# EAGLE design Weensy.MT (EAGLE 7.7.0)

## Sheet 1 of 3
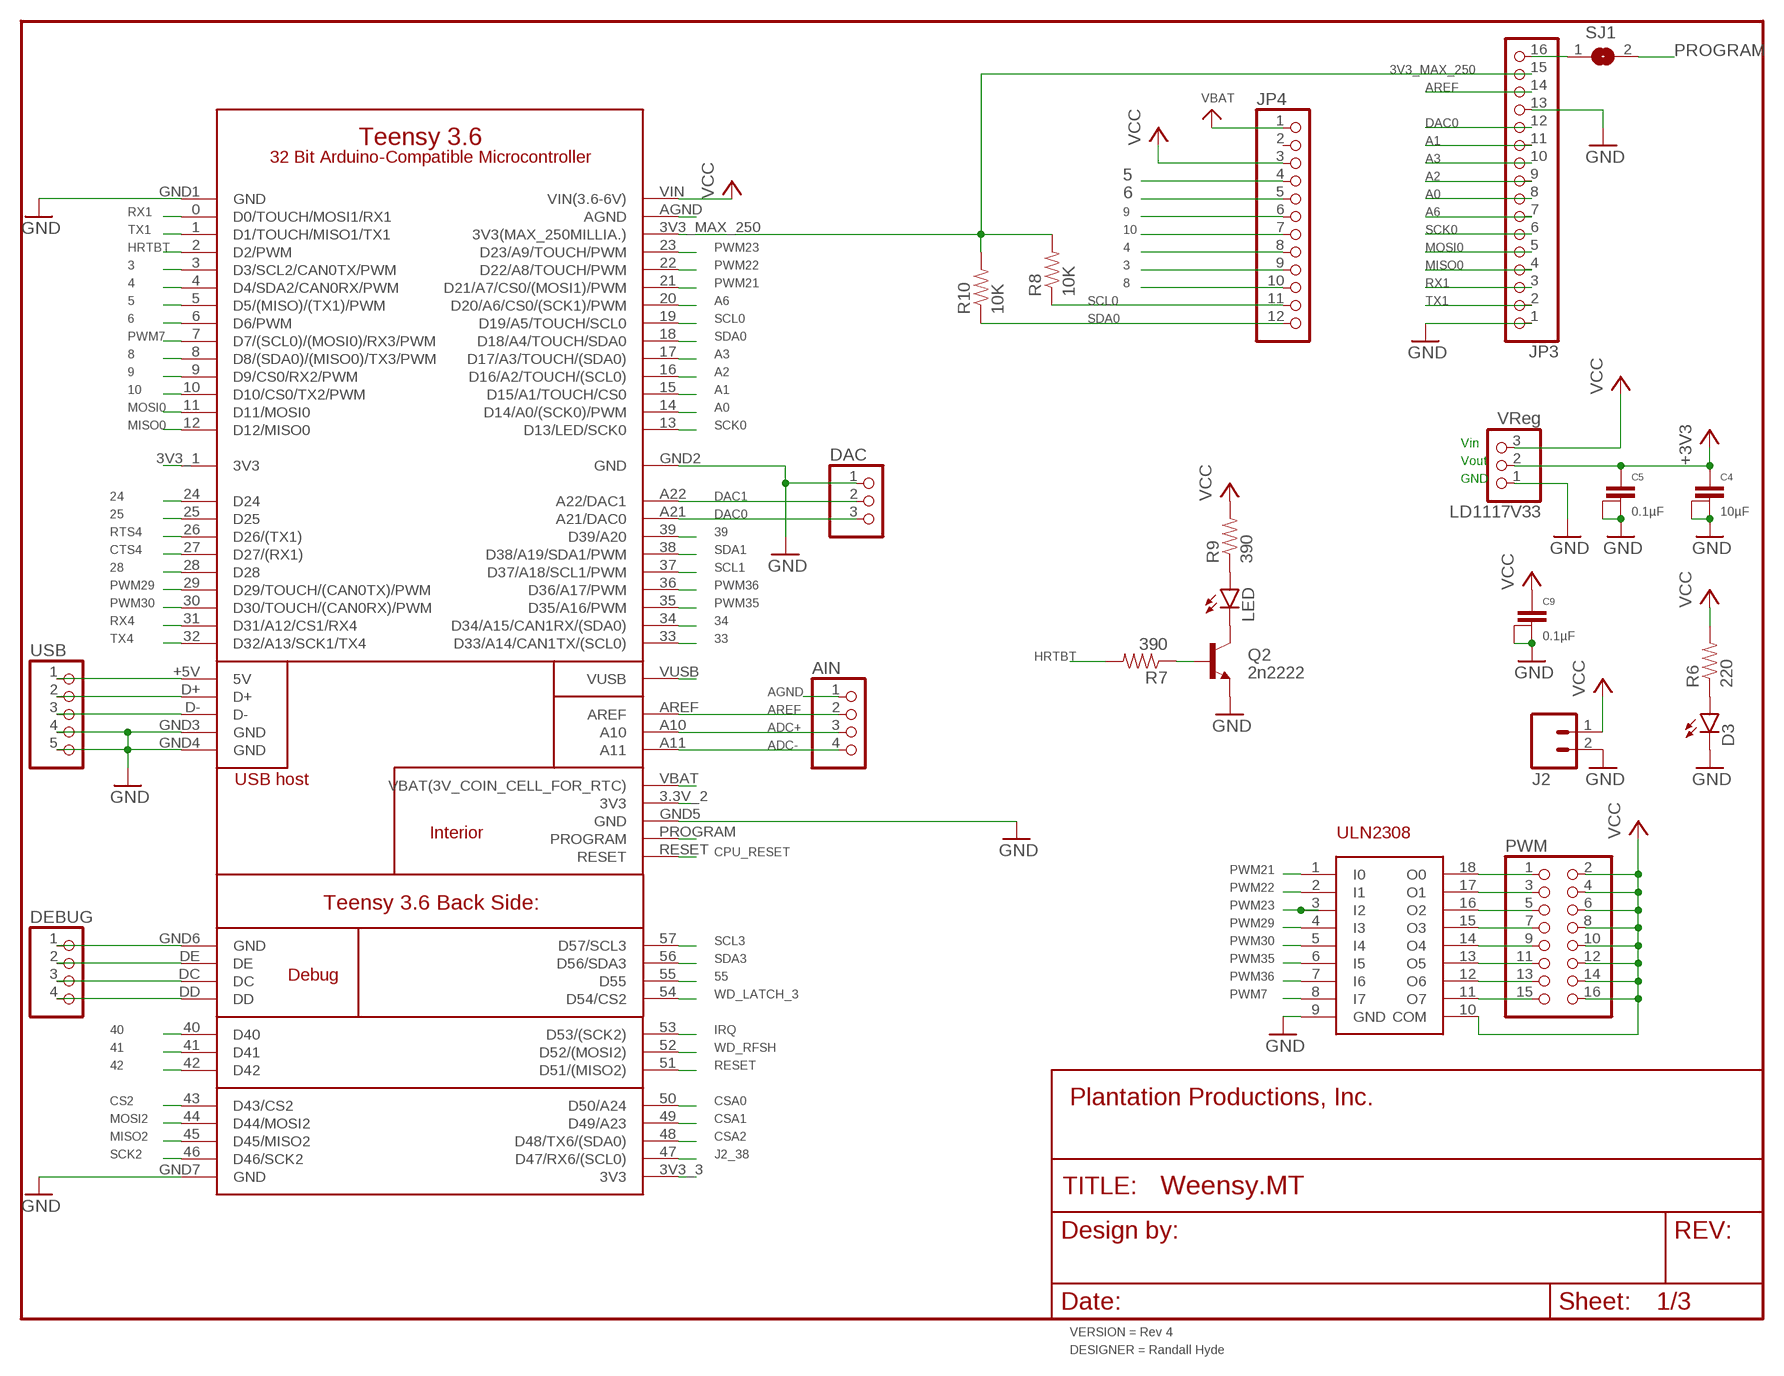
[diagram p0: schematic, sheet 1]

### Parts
AIN  PINHD-1X4  [1X04]
C4  10µF  CAPACITOR  [1+2CAP]
C5  0.1µF  CAPACITOR  [1+2CAP]
C9  0.1µF  CAPACITOR  [1+2CAP]
D3  LED5MM  [LED5MM]
DAC  PINHD-1X3  [1X03]
DEBUG  PINHD-1X4  [1X04]
FRAME1  FRAME-LETTERNO_PACKAGE  [DUMMY]
J2  M025MM  [SCREWTERMINAL-5MM-2]
JP3  HEADER-1X16ROUND  [1X16_ROUND]
JP4  HEADER-1X12  [1X12_ROUND]
LD1117V33  VReg  PINHD-1X3  [1X03]
LED  LED5MM  [LED5MM]
PWM  PINHD-2X8  [2X08]
Q2  2n2222  TRANSISTOR_NPNP2N2222A  [TO-92]
R6  220  1KOHM-1/4W-1%(PTH)  [AXIAL-0.3]
R7  390  10KOHM-1/4W-1%(PTH)HORIZ  [AXIAL-0.3]
R8  10K  10KOHM-1/4W-1%(PTH)HORIZ  [AXIAL-0.3]
R9  390  10KOHM-1/4W-1%(PTH)HORIZ  [AXIAL-0.3]
R10  10K  10KOHM-1/4W-1%(PTH)HORIZ  [AXIAL-0.3]
SJ1  SOLDERJUMPERCLOSED  [SOLDERJUMPER_CLOSEDWIRE]
U$1  TEENSY-3.6_FULL  [TEENSY-3.6_FULL]
ULN2308  ULN2308  [DIL18]
USB  PINHD-1X5  [1X05]

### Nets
3: JP4.9 U$1.3(D3/SCL2/CAN0TX/PWM)
3V3_MAX_250: JP3.15 R8.P$2 R10.P$2 U$1.3V3_MAX_250(3V3(MAX_250MILLIA.))
4: JP4.8 U$1.4(D4/SDA2/CAN0RX/PWM)
5: JP4.4 U$1.5(D5/(MISO)/(TX1)/PWM)
6: JP4.5 U$1.6(D6/PWM)
8: JP4.10 U$1.8(D8/(SDA0)/(MISO0)/TX3/PWM)
9: JP4.6 U$1.9(D9/CS0/RX2/PWM)
10: JP4.7 U$1.10(D10/CS0/TX2/PWM)
24: U$1.24(D24) ; also sheet 2
25: U$1.25(D25) ; also sheet 2
28: U$1.28(D28) ; also sheet 2
33: U$1.33(D33/A14/CAN1TX/(SCL0)) ; also sheet 2
34: U$1.34(D34/A15/CAN1RX/(SDA0)) ; also sheet 2
39: U$1.39(D39/A20) ; also sheet 2
40: U$1.40(D40) ; also sheet 2
41: U$1.41(D41) ; also sheet 2
42: U$1.42(D42) ; also sheet 2
55: U$1.55(D55) ; also sheet 2
+3V3 [Power]: C4.1 C5.1 LD1117V33.2 ; also sheet 2,3
A0: JP3.8 U$1.14(D14/A0/(SCK0)/PWM)
A1: JP3.11 U$1.15(D15/A1/TOUCH/CS0)
A2: JP3.9 U$1.16(D16/A2/TOUCH/(SCL0))
A3: JP3.10 U$1.17(D17/A3/TOUCH/(SDA0))
A6: JP3.7 U$1.20(D20/A6/CS0/(SCK1)/PWM)
ADC+: AIN.3 U$1.A10
ADC-: AIN.4 U$1.A11
AGND: AIN.1 U$1.AGND
AREF: AIN.2 JP3.14 U$1.AREF
CPU_RESET: U$1.RESET
CS2: U$1.43(D43/CS2) ; also sheet 3
CSA0: U$1.50(D50/A24) ; also sheet 3
CSA1: U$1.49(D49/A23) ; also sheet 3
CSA2: U$1.48(D48/TX6/(SDA0)) ; also sheet 3
CTS4: U$1.27(D27/(RX1)) ; also sheet 3
DAC0: DAC.3 JP3.12 U$1.A21(A21/DAC0)
DAC1: DAC.2 U$1.A22(A22/DAC1)
GND: C4.2@1 C4.2@2 C5.2@1 C5.2@2 C9.2@1 C9.2@2 D3.K(C) DAC.1 DEBUG.1 J2.2 JP3.1 JP3.13 LD1117V33.1 Q2.3(E) U$1.GND1(GND) U$1.GND2(GND) U$1.GND3(GND) U$1.GND4(GND) U$1.GND5(GND) U$1.GND6(GND) U$1.GND7(GND) ULN2308.9(GND) USB.4 USB.5 ; also sheet 2,3
HRTBT: R7.P$2 U$1.2(D2/PWM)
IRQ: U$1.53(D53/(SCK2)) ; also sheet 2
J2_38: U$1.47(D47/RX6/(SCL0)) ; also sheet 2
MISO0: JP3.4 U$1.12(D12/MISO0)
MISO2: U$1.45(D45/MISO2) ; also sheet 2
MOSI0: JP3.5 U$1.11(D11/MOSI0)
MOSI2: U$1.44(D44/MOSI2) ; also sheet 2
N$2: D3.A R6.P$1
N$20 [Power]: U$1.3V3_3(3V3)
N$23 [Hi Current]: PWM.1 ULN2308.18(O0)
N$24 [Hi Current]: PWM.3 ULN2308.17(O1)
N$25 [Hi Current]: PWM.5 ULN2308.16(O2)
N$26 [Hi Current]: PWM.7 ULN2308.15(O3)
N$27 [Hi Current]: PWM.9 ULN2308.14(O4)
N$28 [Hi Current]: PWM.11 ULN2308.13(O5)
N$29 [Hi Current]: PWM.13 ULN2308.12(O6)
N$30 [Hi Current]: PWM.15 ULN2308.11(O7)
N$31: U$1.3V3_1(3V3)
N$36: LED.K(C) Q2.1(C)
N$37: Q2.2(B) R7.P$1
N$38: LED.A R9.P$1
N$41: U$1.+5V(5V) USB.1
N$42: U$1.D+ USB.2
N$43: U$1.D- USB.3
N$46: DEBUG.2 U$1.DE
N$47: DEBUG.3 U$1.DC
N$48: DEBUG.4 U$1.DD
N$71: U$1.3.3V_2(3V3)
PROGRAM: SJ1.2 U$1.PROGRAM
PWM7: U$1.7(D7/(SCL0)/(MOSI0)/RX3/PWM) ULN2308.8(I7)
PWM21: U$1.21(D21/A7/CS0/(MOSI1)/PWM) ULN2308.1(I0)
PWM22: U$1.22(D22/A8/TOUCH/PWM) ULN2308.2(I1)
PWM23: U$1.23(D23/A9/TOUCH/PWM) ULN2308.3(I2)
PWM29: U$1.29(D29/TOUCH/(CAN0TX)/PWM) ULN2308.4(I3)
PWM30: U$1.30(D30/TOUCH/(CAN0RX)/PWM) ULN2308.5(I4)
PWM35: U$1.35(D35/A16/PWM) ULN2308.6(I5)
PWM36: U$1.36(D36/A17/PWM) ULN2308.7(I6)
RESET: U$1.51(D51/(MISO2)) ; also sheet 2,3
RST/BOOT: JP3.16 SJ1.1
RTS4: U$1.26(D26/(TX1)) ; also sheet 3
RX1: JP3.3 U$1.0(D0/TOUCH/MOSI1/RX1)
RX4: U$1.31(D31/A12/CS1/RX4) ; also sheet 3
SCK0: JP3.6 U$1.13(D13/LED/SCK0)
SCK2: U$1.46(D46/SCK2) ; also sheet 2,3
SCL0: JP4.11 R8.P$1 U$1.19(D19/A5/TOUCH/SCL0)
SCL1: U$1.37(D37/A18/SCL1/PWM) ; also sheet 2
SCL3: U$1.57(D57/SCL3) ; also sheet 2
SDA0: JP4.12 R10.P$1 U$1.18(D18/A4/TOUCH/SDA0)
SDA1: U$1.38(D38/A19/SDA1/PWM) ; also sheet 2
SDA3: U$1.56(D56/SDA3) ; also sheet 2
TX1: JP3.2 U$1.1(D1/TOUCH/MISO1/TX1)
TX4: U$1.32(D32/A13/SCK1/TX4) ; also sheet 3
VBAT: JP4.1 U$1.VBAT(VBAT(3V_COIN_CELL_FOR_RTC))
VCC [Hi Current]: C9.1 J2.1 JP4.3 LD1117V33.3 PWM.2 PWM.4 PWM.6 PWM.8 PWM.10 PWM.12 PWM.14 PWM.16 R6.P$2 R9.P$2 U$1.VIN(VIN(3.6-6V)) ULN2308.10(COM) ; also sheet 2,3
VUSB: U$1.VUSB
WD_LATCH_3: U$1.54(D54/CS2) ; also sheet 2
WD_RFSH: U$1.52(D52/(MOSI2)) ; also sheet 2
Unconnected: JP4.2

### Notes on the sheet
- Vin
- Vout
- GND

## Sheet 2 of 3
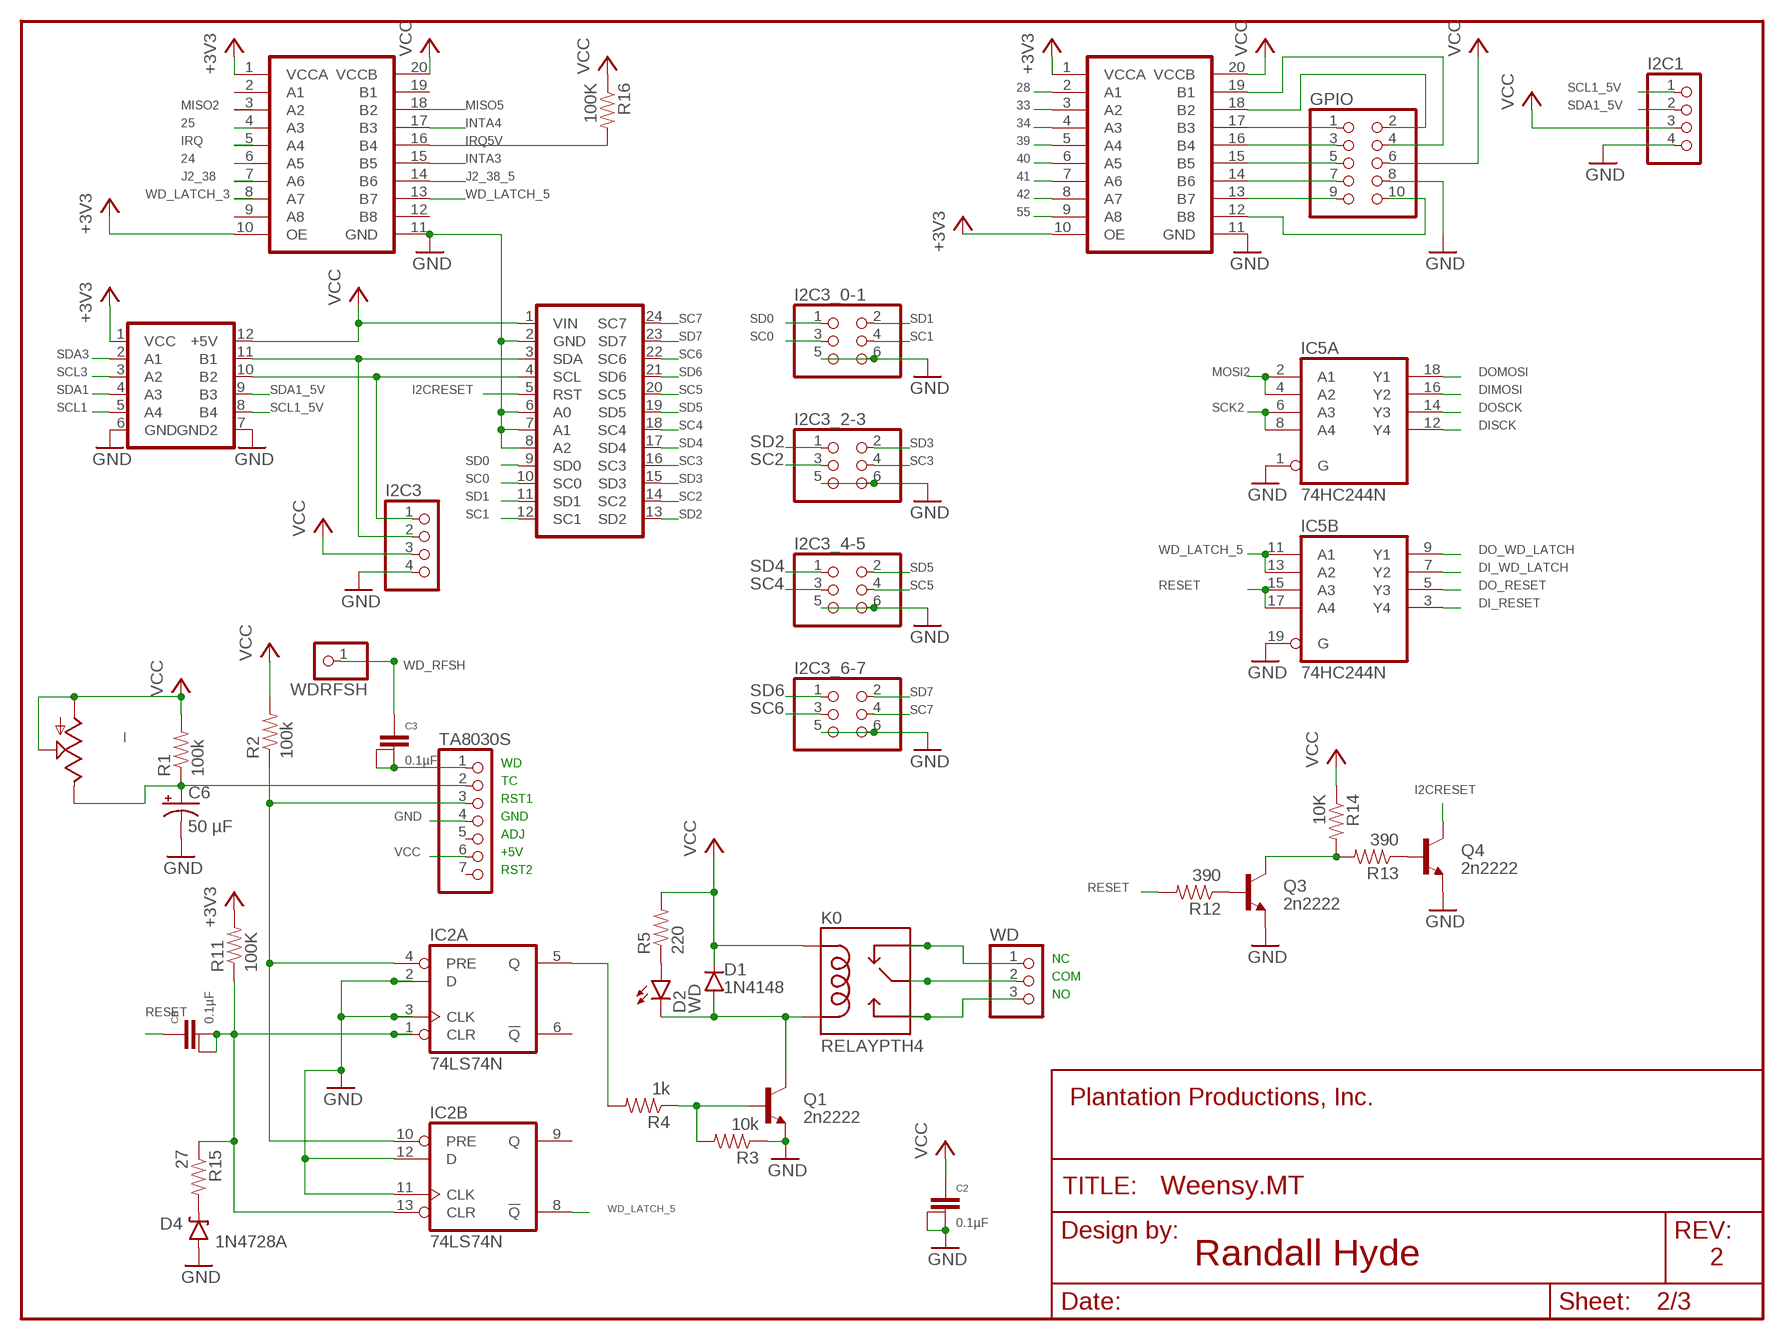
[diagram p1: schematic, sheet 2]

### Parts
_  TRIM_US-B64Y  [B64Y]
BOB1  ADAFRTTXB0108  [DIL20W]
BOB2  ADAFRTBSS138  [DIL12W]
BOB3  ADAFRTTCA9584  [DIL24W]
BOB4  ADAFRTTXB0108  [DIL20W]
C2  0.1µF  CAPACITOR  [1+2CAP]
C3  0.1µF  CAPACITOR  [1+2CAP]
C6  50 µF  100UF-25V-20%(PTH)  [CPOL-RADIAL-100UF-25V]
C8  0.1µF  CAPACITOR  [1+2CAP]
D1  1N4148  DIODE1N4148  [DIODE-1N4148]
D2  WD  LED5MM  [LED5MM]
D4  1N4728A  DIODE-ZENERPTH  [DIODE-ZENER]
FRAME2  FRAME-LETTERNO_PACKAGE  [DUMMY]
GPIO  PINHD-2X5  [2X05]
I2C1  PINHD-1X4  [1X04]
I2C3  PINHD-1X4  [1X04]
I2C3_0-1  PINHD-2X3  [2X03]
I2C3_2-3  PINHD-2X3  [2X03]
I2C3_4-5  PINHD-2X3  [2X03]
I2C3_6-7  PINHD-2X3  [2X03]
IC2  74LS74N  [DIL14]
IC5  74HC244N  [DIL20]
K0  RELAYPTH4  [RELAY-JZC]
Q1  2n2222  TRANSISTOR_NPNP2N2222A  [TO-92]
Q3  2n2222  TRANSISTOR_NPNP2N2222A  [TO-92]
Q4  2n2222  TRANSISTOR_NPNP2N2222A  [TO-92]
R1  100k  10KOHM-1/4W-1%(PTH)HORIZ  [AXIAL-0.3]
R2  100k  10KOHM-1/4W-1%(PTH)HORIZ  [AXIAL-0.3]
R3  10k  10KOHM-1/4W-1%(PTH)HORIZ  [AXIAL-0.3]
R4  1k  10KOHM-1/4W-1%(PTH)HORIZ  [AXIAL-0.3]
R5  220  10KOHM-1/4W-1%(PTH)HORIZ  [AXIAL-0.3]
R11  100K  1KOHM-1/4W-1%(PTH)  [AXIAL-0.3]
R12  390  10KOHM-1/4W-1%(PTH)HORIZ  [AXIAL-0.3]
R13  390  10KOHM-1/4W-1%(PTH)HORIZ  [AXIAL-0.3]
R14  10K  10KOHM-1/4W-1%(PTH)HORIZ  [AXIAL-0.3]
R15  27  1KOHM-1/4W-1%(PTH)  [AXIAL-0.3]
R16  100K  10KOHM-1/4W-1%(PTH)HORIZ  [AXIAL-0.3]
TA8030S  PINHD-1X7  [1X07]
WD  PINHD-1X3  [1X03]
WDRFSH  PINHD-1X1  [1X01]

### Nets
24: BOB1.6(A5) ; also sheet 1
25: BOB1.4(A3) ; also sheet 1
28: BOB4.2(A1) ; also sheet 1
33: BOB4.3(A2) ; also sheet 1
34: BOB4.4(A3) ; also sheet 1
39: BOB4.5(A4) ; also sheet 1
40: BOB4.6(A5) ; also sheet 1
41: BOB4.7(A6) ; also sheet 1
42: BOB4.8(A7) ; also sheet 1
55: BOB4.9(A8) ; also sheet 1
+3V3 [Power]: BOB1.1(VCCA) BOB1.10(OE) BOB2.1(VCC) BOB4.1(VCCA) BOB4.10(OE) R11.P$2 ; also sheet 1,3
DI_RESET: IC5.3(B:Y4) ; also sheet 3
DI_WD_LATCH: IC5.7(B:Y2) ; also sheet 3
DIMOSI: IC5.16(A:Y2) ; also sheet 3
DISCK: IC5.12(A:Y4) ; also sheet 3
DO_RESET: IC5.5(B:Y3) ; also sheet 3
DO_WD_LATCH: IC5.9(B:Y1) ; also sheet 3
DOMOSI: IC5.18(A:Y1) ; also sheet 3
DOSCK: IC5.14(A:Y3) ; also sheet 3
GND: BOB1.11(GND) BOB2.6(GND) BOB2.7(GND2) BOB3.2(GND) BOB3.6(A0) BOB3.7(A1) BOB3.8(A2) BOB4.11(GND) C2.2@1 C2.2@2 C6.2(-) D4.P$2(A) GPIO.8 I2C1.4 I2C3.4 I2C3_0-1.5 I2C3_0-1.6 I2C3_2-3.5 I2C3_2-3.6 I2C3_4-5.5 I2C3_4-5.6 I2C3_6-7.5 I2C3_6-7.6 IC2.2(A:D) IC2.3(A:CLK) IC2.11(B:CLK) IC2.12(B:D) IC5.1(A:G) IC5.19(B:G) Q1.3(E) Q3.3(E) Q4.3(E) R3.P$1 TA8030S.4 ; also sheet 1,3
GPIO28: BOB4.19(B1) GPIO.4
GPIO33: BOB4.18(B2) GPIO.2
GPIO34: BOB4.17(B3) GPIO.1
GPIO39: BOB4.16(B4) GPIO.3
GPIO40: BOB4.15(B5) GPIO.5
GPIO41: BOB4.14(B6) GPIO.7
GPIO42: BOB4.13(B7) GPIO.9
GPIO55: BOB4.12(B8) GPIO.10
I2CRESET: BOB3.5(RST) Q4.1(C)
INTA3: BOB1.15(B5) ; also sheet 3
INTA4: BOB1.17(B3) ; also sheet 3
IRQ: BOB1.5(A4) ; also sheet 1
IRQ5V: BOB1.16(B4) R16.P$2 ; also sheet 3
J2_38: BOB1.7(A6) ; also sheet 1
J2_38_5: BOB1.14(B6) ; also sheet 3
MISO2: BOB1.3(A2) ; also sheet 1
MISO5: BOB1.18(B2) ; also sheet 3
MOSI2: IC5.2(A:A1) IC5.4(A:A2) ; also sheet 1
N$3: C3.2@1 C3.2@2 TA8030S.1
N$4: _.E C6.1(+) R1.P$1 TA8030S.2
N$5: BOB2.11(B1) BOB3.3(SDA) I2C3.2
N$6: D1.A D2.K(C) K0.1(COIL2) Q1.1(C)
N$9: D2.A R5.P$1
N$11: Q1.2(B) R3.P$2 R4.P$1
N$12: Q3.2(B) R12.P$1
N$13: Q4.2(B) R13.P$1
N$14 [Power]: K0.4(MAIN) WD.2
N$15 [Power]: K0.3(NO) WD.3
N$16: BOB2.10(B2) BOB3.4(SCL) I2C3.1
N$17: Q3.1(C) R13.P$2 R14.P$2
N$39: D4.P$1(C) R15.P$2
NC [Power]: K0.2(NC) WD.1
RESET: C8.1 IC5.15(B:A3) IC5.17(B:A4) R12.P$2 ; also sheet 1,3
RESETWD: C8.2@1 C8.2@2 IC2.1(A:CLR) IC2.13(B:CLR) R11.P$1 R15.P$1
RST1: IC2.4(A:PRE) IC2.10(B:PRE) R2.P$1 TA8030S.3
SC0: BOB3.10(SC0) I2C3_0-1.3
SC1: BOB3.12(SC1) I2C3_0-1.4
SC2: BOB3.14(SC2) I2C3_2-3.3
SC3: BOB3.16(SC3) I2C3_2-3.4
SC4: BOB3.18(SC4) I2C3_4-5.3
SC5: BOB3.20(SC5) I2C3_4-5.4
SC6: BOB3.22(SC6) I2C3_6-7.3
SC7: BOB3.24(SC7) I2C3_6-7.4
SCK2: IC5.6(A:A3) IC5.8(A:A4) ; also sheet 1,3
SCL1: BOB2.5(A4) ; also sheet 1
SCL1_5V: BOB2.8(B4) I2C1.1
SCL3: BOB2.3(A2) ; also sheet 1
SD0: BOB3.9(SD0) I2C3_0-1.1
SD1: BOB3.11(SD1) I2C3_0-1.2
SD2: BOB3.13(SD2) I2C3_2-3.1
SD3: BOB3.15(SD3) I2C3_2-3.2
SD4: BOB3.17(SD4) I2C3_4-5.1
SD5: BOB3.19(SD5) I2C3_4-5.2
SD6: BOB3.21(SD6) I2C3_6-7.1
SD7: BOB3.23(SD7) I2C3_6-7.2
SDA1: BOB2.4(A3) ; also sheet 1
SDA1_5V: BOB2.9(B3) I2C1.2
SDA3: BOB2.2(A1) ; also sheet 1
VCC [Hi Current]: _.A _.S BOB1.20(VCCB) BOB2.12(+5V) BOB3.1(VIN) BOB4.20(VCCB) C2.1 D1.C GPIO.6 I2C1.3 I2C3.3 K0.5(COIL1) R1.P$2 R2.P$2 R5.P$2 R14.P$1 R16.P$1 TA8030S.6 ; also sheet 1,3
WD_LATCH_3: BOB1.8(A7) ; also sheet 1
WD_LATCH_5: BOB1.13(B7) IC2.8(B:!Q) IC5.11(B:A1) IC5.13(B:A2)
WD_RFSH: C3.1 WDRFSH.1 ; also sheet 1
WDOUT: IC2.5(A:Q) R4.P$2
Unconnected: BOB1.2(A1) BOB1.9(A8) BOB1.12(B8) BOB1.19(B1) IC2.6(A:!Q) IC2.9(B:Q) TA8030S.5 TA8030S.7

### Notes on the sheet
- WD
- TC
- RST1
- GND
- ADJ
- +5V
- RST2
- NC
- COM
- NO
- Randall Hyde | 2

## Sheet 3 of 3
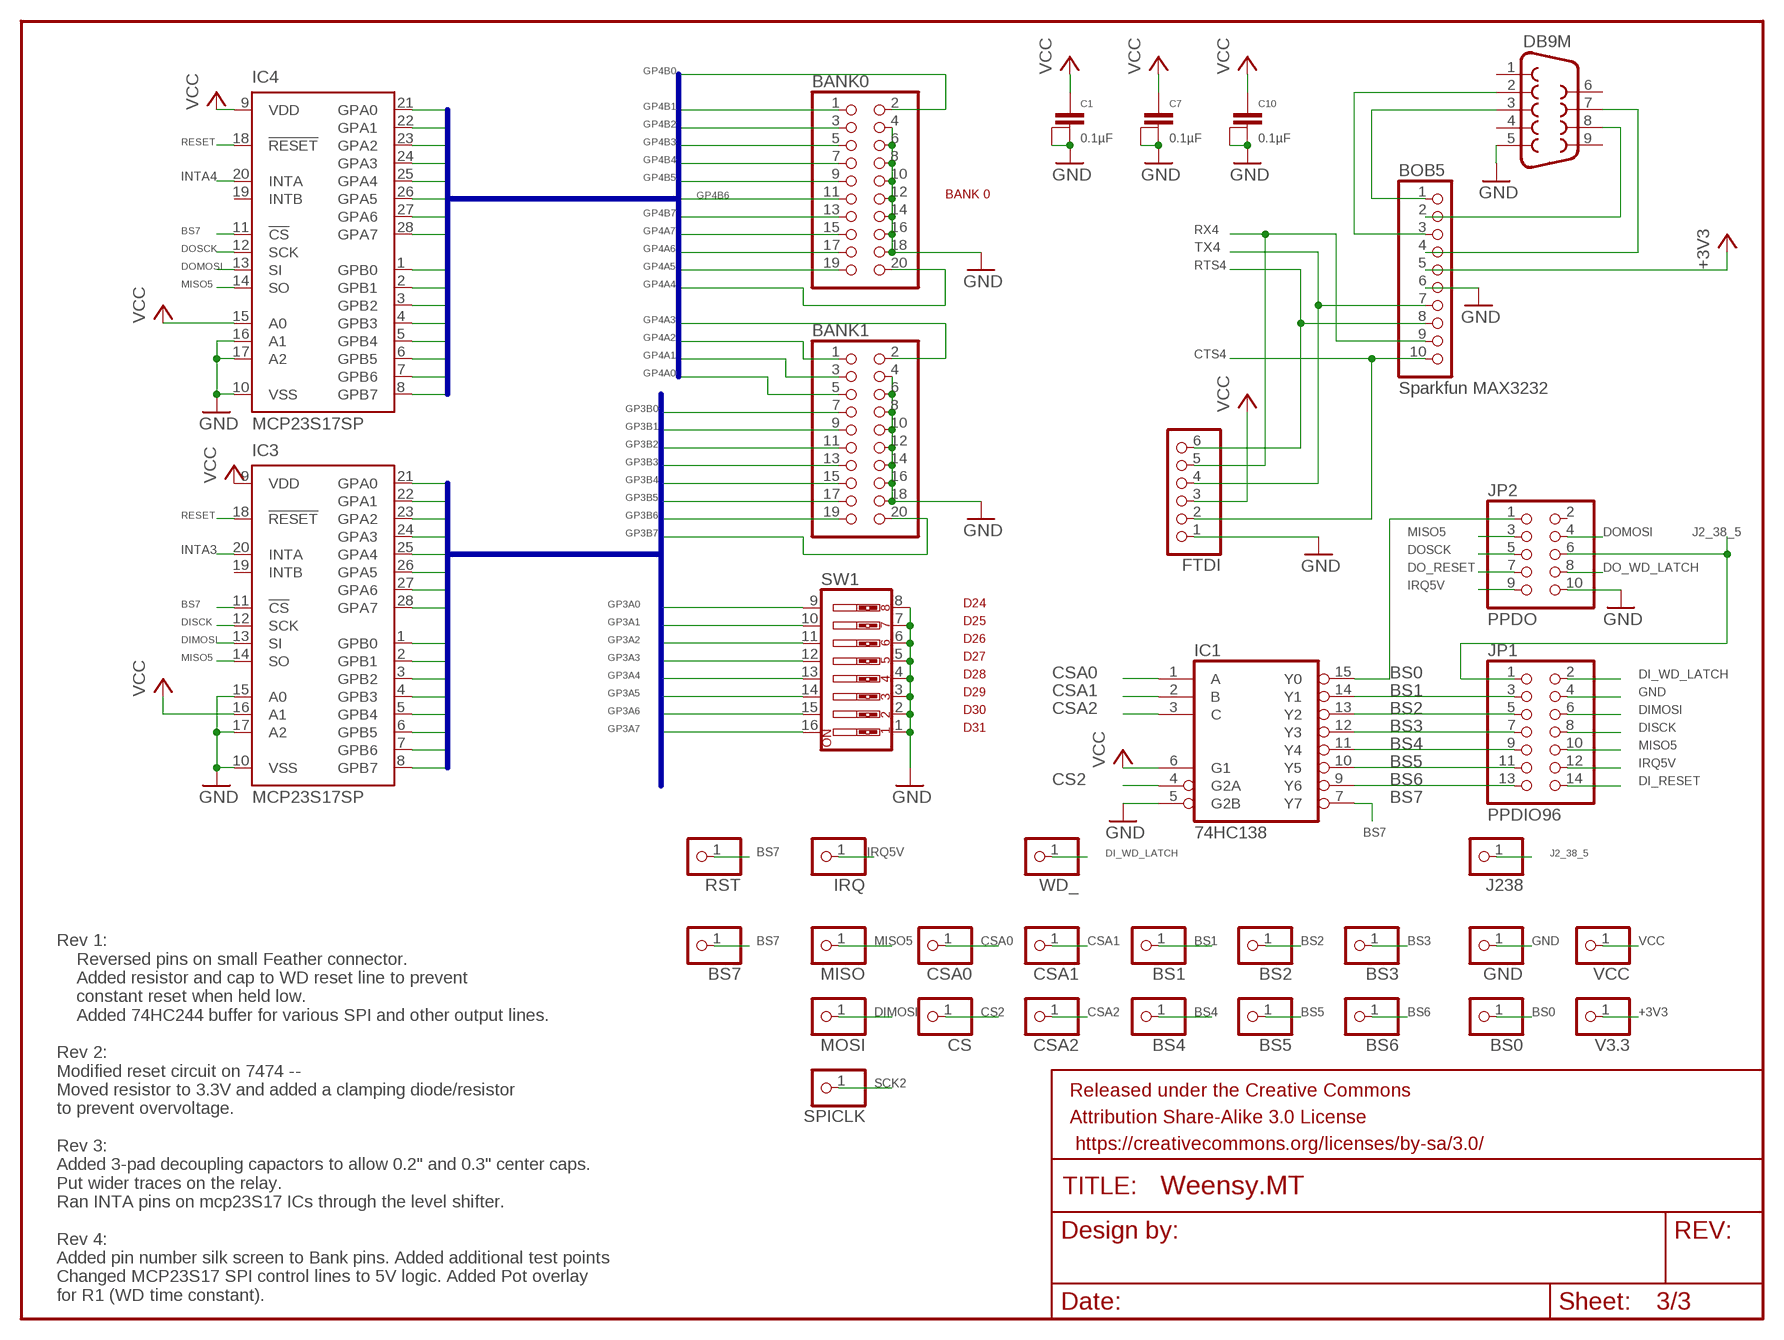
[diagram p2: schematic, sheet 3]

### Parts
BANK0  PINHD-2X10  [2X10]
BANK1  PINHD-2X10  [2X10]
BOB5  Sparkfun MAX3232  PINHD-1X10  [1X10]
BS0  PINHD-1X1  [1X01]
BS1  PINHD-1X1  [1X01]
BS2  PINHD-1X1  [1X01]
BS3  PINHD-1X1  [1X01]
BS4  PINHD-1X1  [1X01]
BS5  PINHD-1X1  [1X01]
BS6  PINHD-1X1  [1X01]
BS7  PINHD-1X1  [1X01]
C1  0.1µF  CAPACITOR  [1+2CAP]
C7  0.1µF  CAPACITOR  [1+2CAP]
C10  0.1µF  CAPACITOR  [1+2CAP]
CS  PINHD-1X1  [1X01]
CSA0  PINHD-1X1  [1X01]
CSA1  PINHD-1X1  [1X01]
CSA2  PINHD-1X1  [1X01]
DB9M  DB9MALE  [DB9_MALE]
FRAME3  FRAME-LETTER  [CREATIVE_COMMONS]
FTDI  PINHD-1X6  [1X06]
GND  PINHD-1X1  [1X01]
IC1  74HC138  74LS138N  [DIL16]
IC3  MCP23S17SP  [DIL28-3]
IC4  MCP23S17SP  [DIL28-3]
IRQ  PINHD-1X1  [1X01]
J238  PINHD-1X1  [1X01]
JP1  PPDIO96  PINHD-2X7  [2X07]
JP2  PPDO  PINHD-2X5  [2X05]
MISO  PINHD-1X1  [1X01]
MOSI  PINHD-1X1  [1X01]
RST  PINHD-1X1  [1X01]
SPICLK  PINHD-1X1  [1X01]
SW1  SW_DIP-8  [DIPSWITCH-08]
V3.3  PINHD-1X1  [1X01]
VCC  PINHD-1X1  [1X01]
WD_  PINHD-1X1  [1X01]

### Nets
+3V3 [Power]: BOB5.5 V3.3.1 ; also sheet 1,2
BS0: BS0.1 IC1.15(Y0) JP2.1
BS1: BS1.1 IC1.14(Y1) JP1.3
BS2: BS2.1 IC1.13(Y2) JP1.5
BS3: BS3.1 IC1.12(Y3) JP1.7
BS4: BS4.1 IC1.11(Y4) JP1.9
BS5: BS5.1 IC1.10(Y5) JP1.11
BS6: BS6.1 IC1.9(Y6) JP1.13
BS7: BS7.1 IC1.7(Y7) IC3.11(!CS) IC4.11(!CS) RST.1
CS2: CS.1 IC1.4(G2A) ; also sheet 1
CSA0: CSA0.1 IC1.1(A) ; also sheet 1
CSA1: CSA1.1 IC1.2(B) ; also sheet 1
CSA2: CSA2.1 IC1.3(C) ; also sheet 1
CTS4: BOB5.10 FTDI.2 ; also sheet 1
DI_RESET: JP1.14 ; also sheet 2
DI_WD_LATCH: JP1.2 WD_.1 ; also sheet 2
DIMOSI: IC3.13(SI) JP1.6 MOSI.1 ; also sheet 2
DISCK: IC3.12(SCK) JP1.8 ; also sheet 2
DO_RESET: JP2.7 ; also sheet 2
DO_WD_LATCH: JP2.8 ; also sheet 2
DOMOSI: IC4.13(SI) JP2.4 ; also sheet 2
DOSCK: IC4.12(SCK) JP2.5 ; also sheet 2
GND: BANK0.4 BANK0.6 BANK0.8 BANK0.10 BANK0.12 BANK0.14 BANK0.16 BANK0.18 BANK1.4 BANK1.6 BANK1.8 BANK1.10 BANK1.12 BANK1.14 BANK1.16 BANK1.18 BOB5.6 C1.2@1 C1.2@2 C7.2@1 C7.2@2 C10.2@1 C10.2@2 DB9M.5 FTDI.1 GND.1 IC1.5(G2B) IC3.10(VSS) IC3.15(A0) IC3.17(A2) IC4.10(VSS) IC4.16(A1) IC4.17(A2) JP1.4 JP2.10 SW1.1 SW1.2 SW1.3 SW1.4 SW1.5 SW1.6 SW1.7 SW1.8 ; also sheet 1,2
GP3A0: IC3.28(GPA7) SW1.9
GP3A1: IC3.27(GPA6) SW1.10
GP3A2: IC3.26(GPA5) SW1.11
GP3A3: IC3.25(GPA4) SW1.12
GP3A4: IC3.24(GPA3) SW1.13
GP3A5: IC3.23(GPA2) SW1.14
GP3A6: IC3.22(GPA1) SW1.15
GP3A7: IC3.21(GPA0) SW1.16
GP3B0: BANK1.7 IC3.1(GPB0)
GP3B1: BANK1.9 IC3.2(GPB1)
GP3B2: BANK1.11 IC3.3(GPB2)
GP3B3: BANK1.13 IC3.4(GPB3)
GP3B4: BANK1.15 IC3.5(GPB4)
GP3B5: BANK1.17 IC3.6(GPB5)
GP3B6: BANK1.19 IC3.7(GPB6)
GP3B7: BANK1.20 IC3.8(GPB7)
GP4A0: BANK1.5 IC4.21(GPA0)
GP4A1: BANK1.3 IC4.22(GPA1)
GP4A2: BANK1.1 IC4.23(GPA2)
GP4A3: BANK1.2 IC4.24(GPA3)
GP4A4: BANK0.20 IC4.25(GPA4)
GP4A5: BANK0.19 IC4.26(GPA5)
GP4A6: BANK0.17 IC4.27(GPA6)
GP4A7: BANK0.15 IC4.28(GPA7)
GP4B0: BANK0.2 IC4.1(GPB0)
GP4B1: BANK0.1 IC4.2(GPB1)
GP4B2: BANK0.3 IC4.3(GPB2)
GP4B3: BANK0.5 IC4.4(GPB3)
GP4B4: BANK0.7 IC4.5(GPB4)
GP4B5: BANK0.9 IC4.6(GPB5)
GP4B6: BANK0.11 IC4.7(GPB6)
GP4B7: BANK0.13 IC4.8(GPB7)
INTA3: IC3.20(INTA) ; also sheet 2
INTA4: IC4.20(INTA) ; also sheet 2
IRQ5V: IRQ.1 JP1.12 JP2.9 ; also sheet 2
J2_38_5: J238.1 JP1.1 JP2.6 ; also sheet 2
MISO5: IC3.14(SO) IC4.14(SO) JP1.10 JP2.3 MISO.1 ; also sheet 2
N$32: BOB5.2 DB9M.8
N$33: BOB5.4 DB9M.7
N$34: BOB5.1 DB9M.3
N$35: BOB5.3 DB9M.2
RESET: IC3.18(!RESET) IC4.18(!RESET) ; also sheet 1,2
RTS4: BOB5.8 FTDI.6 ; also sheet 1
RX4: BOB5.9 FTDI.5 ; also sheet 1
SCK2: SPICLK.1 ; also sheet 1,2
TX4: BOB5.7 FTDI.4 ; also sheet 1
VCC [Hi Current]: C1.1 C7.1 C10.1 FTDI.3 IC1.6(G1) IC3.9(VDD) IC3.16(A1) IC4.9(VDD) IC4.15(A0) VCC.1 ; also sheet 1,2
Unconnected: DB9M.1 DB9M.4 DB9M.6 DB9M.9 IC3.19(INTB) IC4.19(INTB) JP2.2

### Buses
IC2BUS:GP4A[0..7],GP4B[0..7]
IC3BUS:GP3A[0..7],GP3B[0..7]

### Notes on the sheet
- BANK 0
- D24
- D25
- D26
- D27
- D28
- D29
- D30
- D31
- Rev 1:
      Reversed pins on small Feather connector.
      Added resistor and cap to WD reset line to prevent
      constant reset when held low.
      Added 74HC244 buffer for various SPI and other output lines.
  
  Rev 2:
  Modified reset circuit on 7474 -- 
  Moved resistor to 3.3V and added a clamping diode/resistor 
  to prevent overvoltage.
  
  Rev 3:
  Added 3-pad decoupling capactors to allow 0.2" and 0.3" center caps.
  Put wider traces on the relay.
  Ran INTA pins on mcp23S17 ICs through the level shifter.
  
  Rev 4:
  Added pin number silk screen to Bank pins. Added additional test points
  Changed MCP23S17 SPI control lines to 5V logic. Added Pot overlay
  for R1 (WD time constant).

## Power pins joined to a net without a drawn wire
GND: IC1.8(GND) IC2.7(P:GND) IC5.10(P:GND)
VCC: IC1.16(VCC) IC2.14(P:VCC) IC5.20(P:VCC)

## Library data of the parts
_ = pot:TRIM_US-: POTENTIOMETER
AIN DEBUG I2C1 I2C3 = pinhead:PINHD-1X4: PIN HEADER
BANK0 BANK1 = SparkFun-Connectors:PINHD-2X10: PIN HEADER
BOB1 BOB4 = PlantProd:ADAFRTTXB0108: AdaFruit TXB0108 8-channel level shifter
BOB2 = PlantProd:ADAFRTBSS138: AdaFruit BSS138 4-channel I2C bi-directional logical level converter
BOB3 = PlantProd:ADAFRTTCA9584: AdaFruit TCA9548A 8-channel I2C multiplexer
BOB5 = pinhead:PINHD-1X10: PIN HEADER
BS0 BS1-BS7 CS CSA0 CSA1 CSA2 GND IRQ J238 MISO MOSI RST SPICLK V3.3 VCC WD_ WDRFSH = pinhead:PINHD-1X1: PIN HEADER
C1-C5 C7-C10 = PlantProd:CAPACITOR: Capacitor with three terminals to support multiple capacitor sizes.
C6 = SparkFun-Capacitors:100UF-25V-20%(PTH): CAP-08439; PROD_ID: CAP-08439
D1 = SparkFun-DiscreteSemi:DIODE: Diode; PROD_ID: DIO-08378
D2 D3 LED = SparkFun-LED:LED: LEDs
D4 = SparkFun-DiscreteSemi:DIODE-ZENER: Zener Diode
DAC LD1117V33 WD = pinhead:PINHD-1X3: PIN HEADER
DB9M = SparkFun-Connectors:DB9: DB9 Connector Standard DB9 (D-Sub 9) serial connector. Can be used for CAN bus as well as RS485 and RS232. Footprint production proven. Spark Fun Electronics SKU : PRT-00429; PROD_ID: CONN-09904
FRAME1 = SparkFun-Aesthetics:FRAME-LETTER: Schematic Frame; DESIGNER: Randall Hyde; VERSION: Rev 4
FRAME2 = SparkFun-Aesthetics:FRAME-LETTER: Schematic Frame; DESIGNER: Nobody; VERSION: v01
FRAME3 = SparkFun-Retired:FRAME-LETTER: Schematic Frame
FTDI = pinhead:PINHD-1X6: PIN HEADER
GPIO JP2 = pinhead:PINHD-2X5: PIN HEADER
I2C3_0-1 I2C3_2-3 I2C3_4-5 I2C3_6-7 = pinhead:PINHD-2X3: PIN HEADER
IC1 = 74xx-us:74*138: 3-line to 8-line DECODER/DEMULTIPLEXER
IC2 = 74xx-us:74*74: Dual D type positive edge triggered FLIP FLOP, preset and clear
IC3 IC4 = microchip:MCP23S17: http://ww1.microchip.com/downloads/en/DeviceDoc/21952a.pdf Source: http://ww1.microchip.com/downloads/en/DeviceDoc/21952a.pdf; MF: MICROCHIP; MPN: MCP23S17-E/SP; OC_FARNELL: 1292238; OC_NEWARK: 31K2951
IC5 = 74xx-eu:74*244: Octal BUFFER and LINE DRIVER, 3-state
J2 = SparkFun-Connectors:M02: Standard 2-pin 0.1" header. Use with; STOREFRONT_ID: PRT-08432
JP1 = pinhead:PINHD-2X7: PIN HEADER
JP3 = microbuilder:HEADER-1X16: PIN HEADER
JP4 = microbuilder:HEADER-1X12
K0 = SparkFun-Electromechanical:RELAY: SPDT relay (COM-00101)
PWM = pinhead:PINHD-2X8: PIN HEADER
Q1-Q4 = SparkFun-DiscreteSemi:TRANSISTOR_NPN: Generic NPN BJT MMBT2222A - TRANS-08049 (SOT-23, 1A 40V) MPSA42 - TRANS-09116 (SOT-23, 500mA 300V) MMBT5088LT1G - TRANS-11160 (SOT-23, 50 mA 30V) BC547 - COM-08928 (TO-92 45V 100mA) (1.Collector 2.Base 3.Emitter) 2N3904 - COM-00521 (TO-92 40V 200mA) (1.Emitter 2.Base 3.Collector) P2N2222A -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; PROD_ID: TRANS-09536
R1 R2 R4 R5 R7-R10 R12-R14 R16 = SparkFun-Resistors:10KOHM-1/4W-1%(PTH): RES-12183; PROD_ID: RES-12183; VALUE: 10k
R3 = SparkFun-Resistors:10KOHM-1/4W-1%(PTH): RES-12183; PROD_ID: RES-12183
R6 R11 R15 = SparkFun-Resistors:1KOHM-1/4W-1%(PTH): RES-12182; PROD_ID: RES-12182; VALUE: 1K
SJ1 = microbuilder:SOLDERJUMPER: SMD Solder JUMPER
SW1 = SparkFun-Electromechanical:SW_DIP-8: DIP Switch 8 Position
TA8030S = pinhead:PINHD-1X7: PIN HEADER
U$1 = Teensy-3.6:TEENSY-3.6_FULL
ULN2308 = PlantProd:ULN2308: ULN2308 8-Ch Darlington
USB = pinhead:PINHD-1X5: PIN HEADER

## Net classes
1 Power: width 1.016 mm, drill 0.127 mm, clearance 0.254 mm
2 Hi Current: width 0.508 mm, drill 0.254 mm, clearance 0.254 mm
3 Relay: width 2.54 mm, drill 0.254 mm, clearance 0.254 mm

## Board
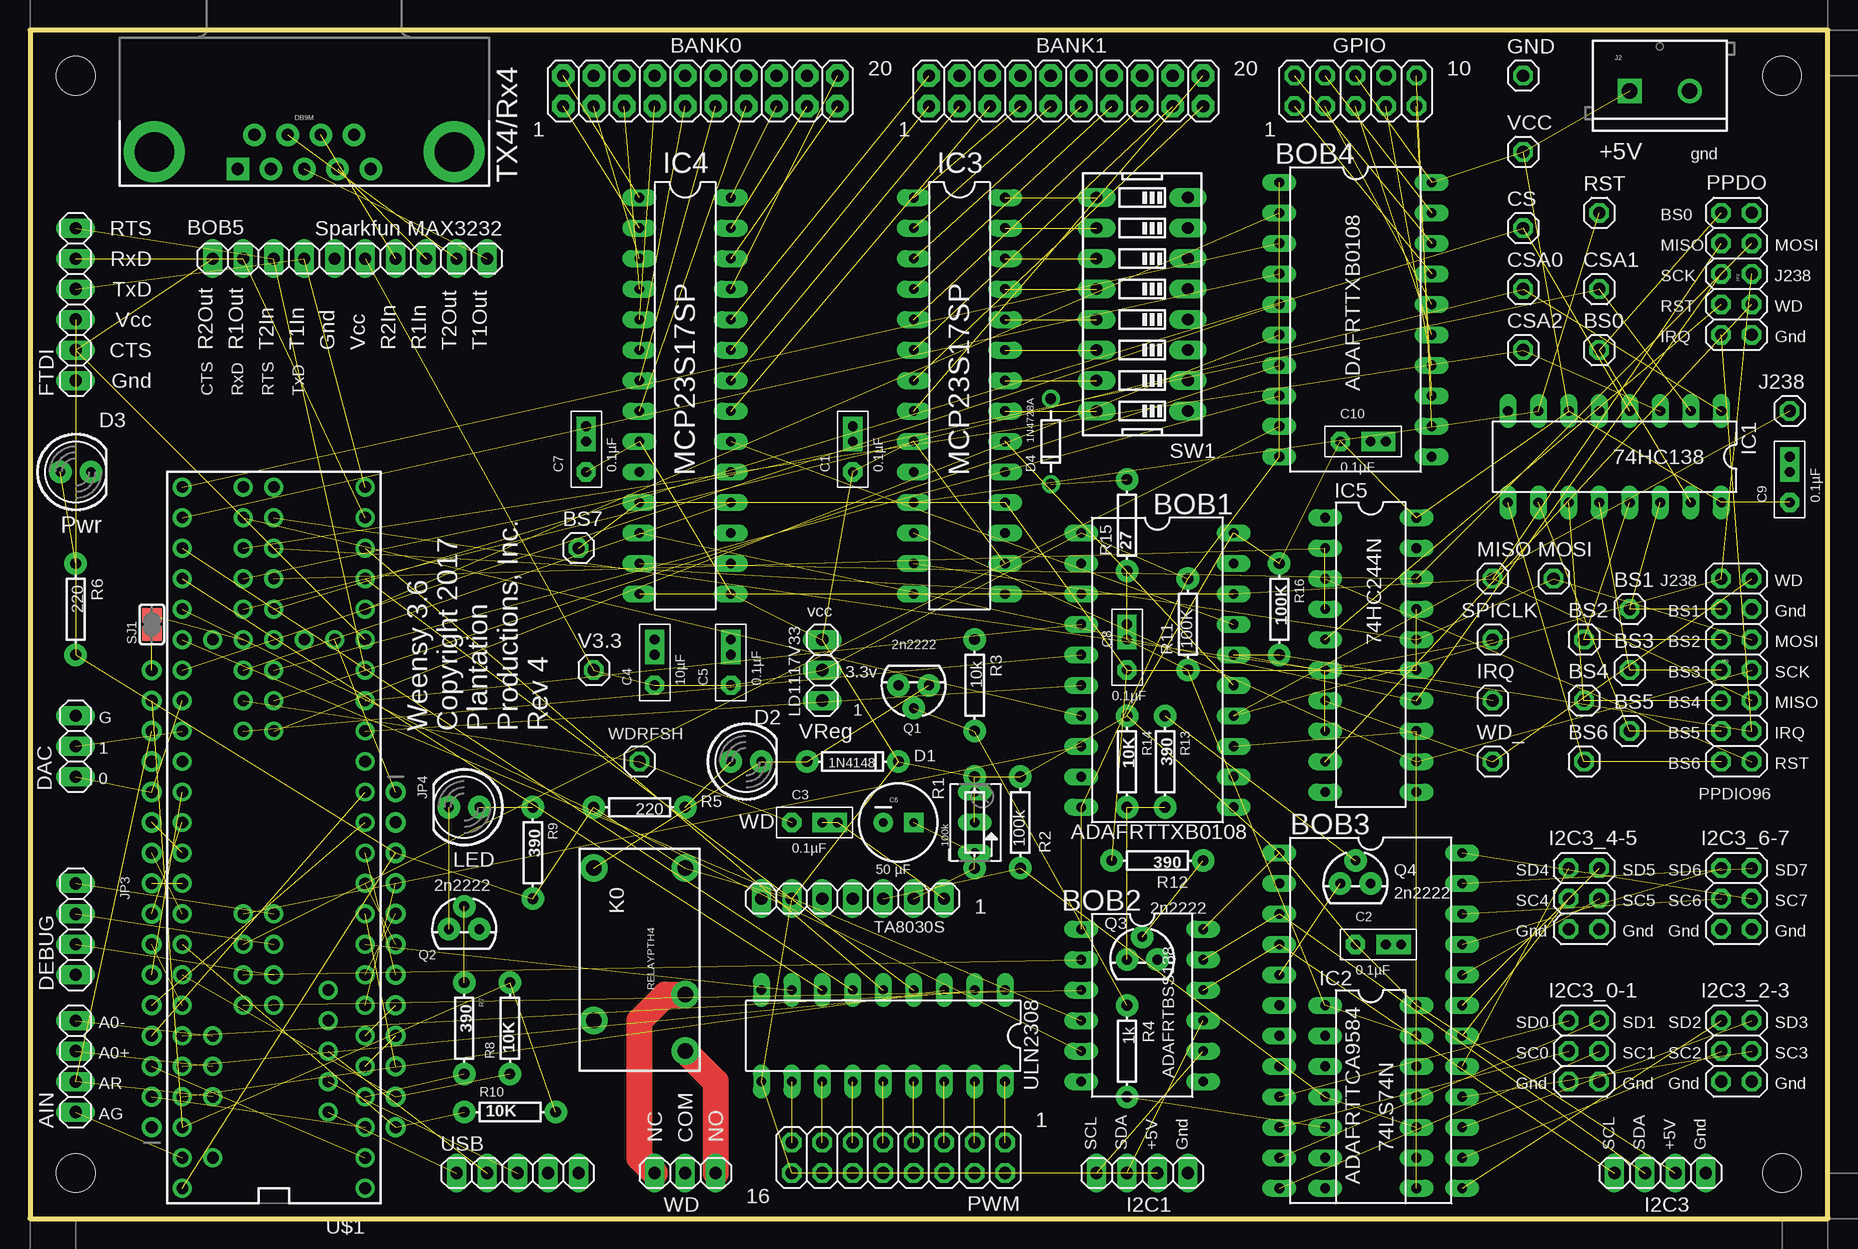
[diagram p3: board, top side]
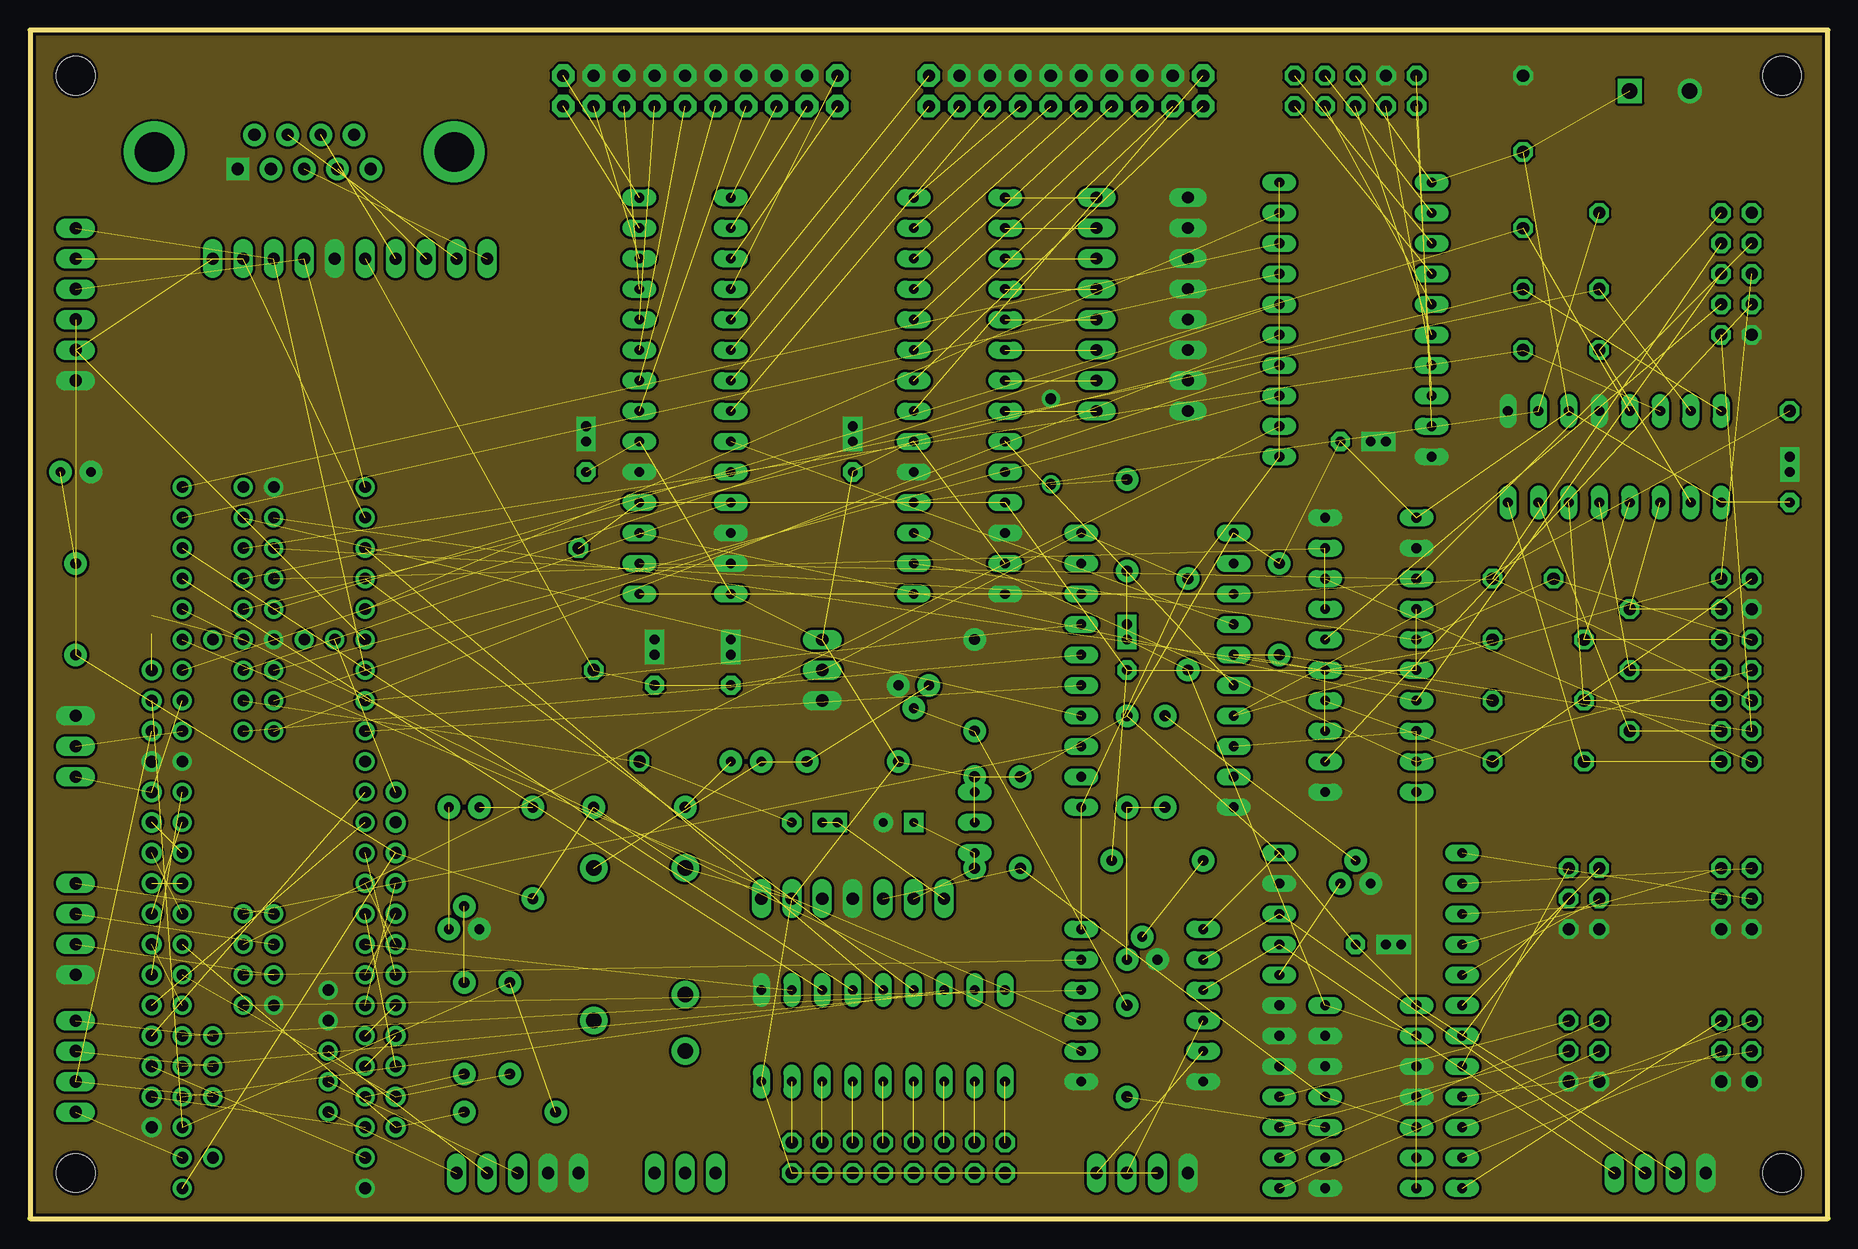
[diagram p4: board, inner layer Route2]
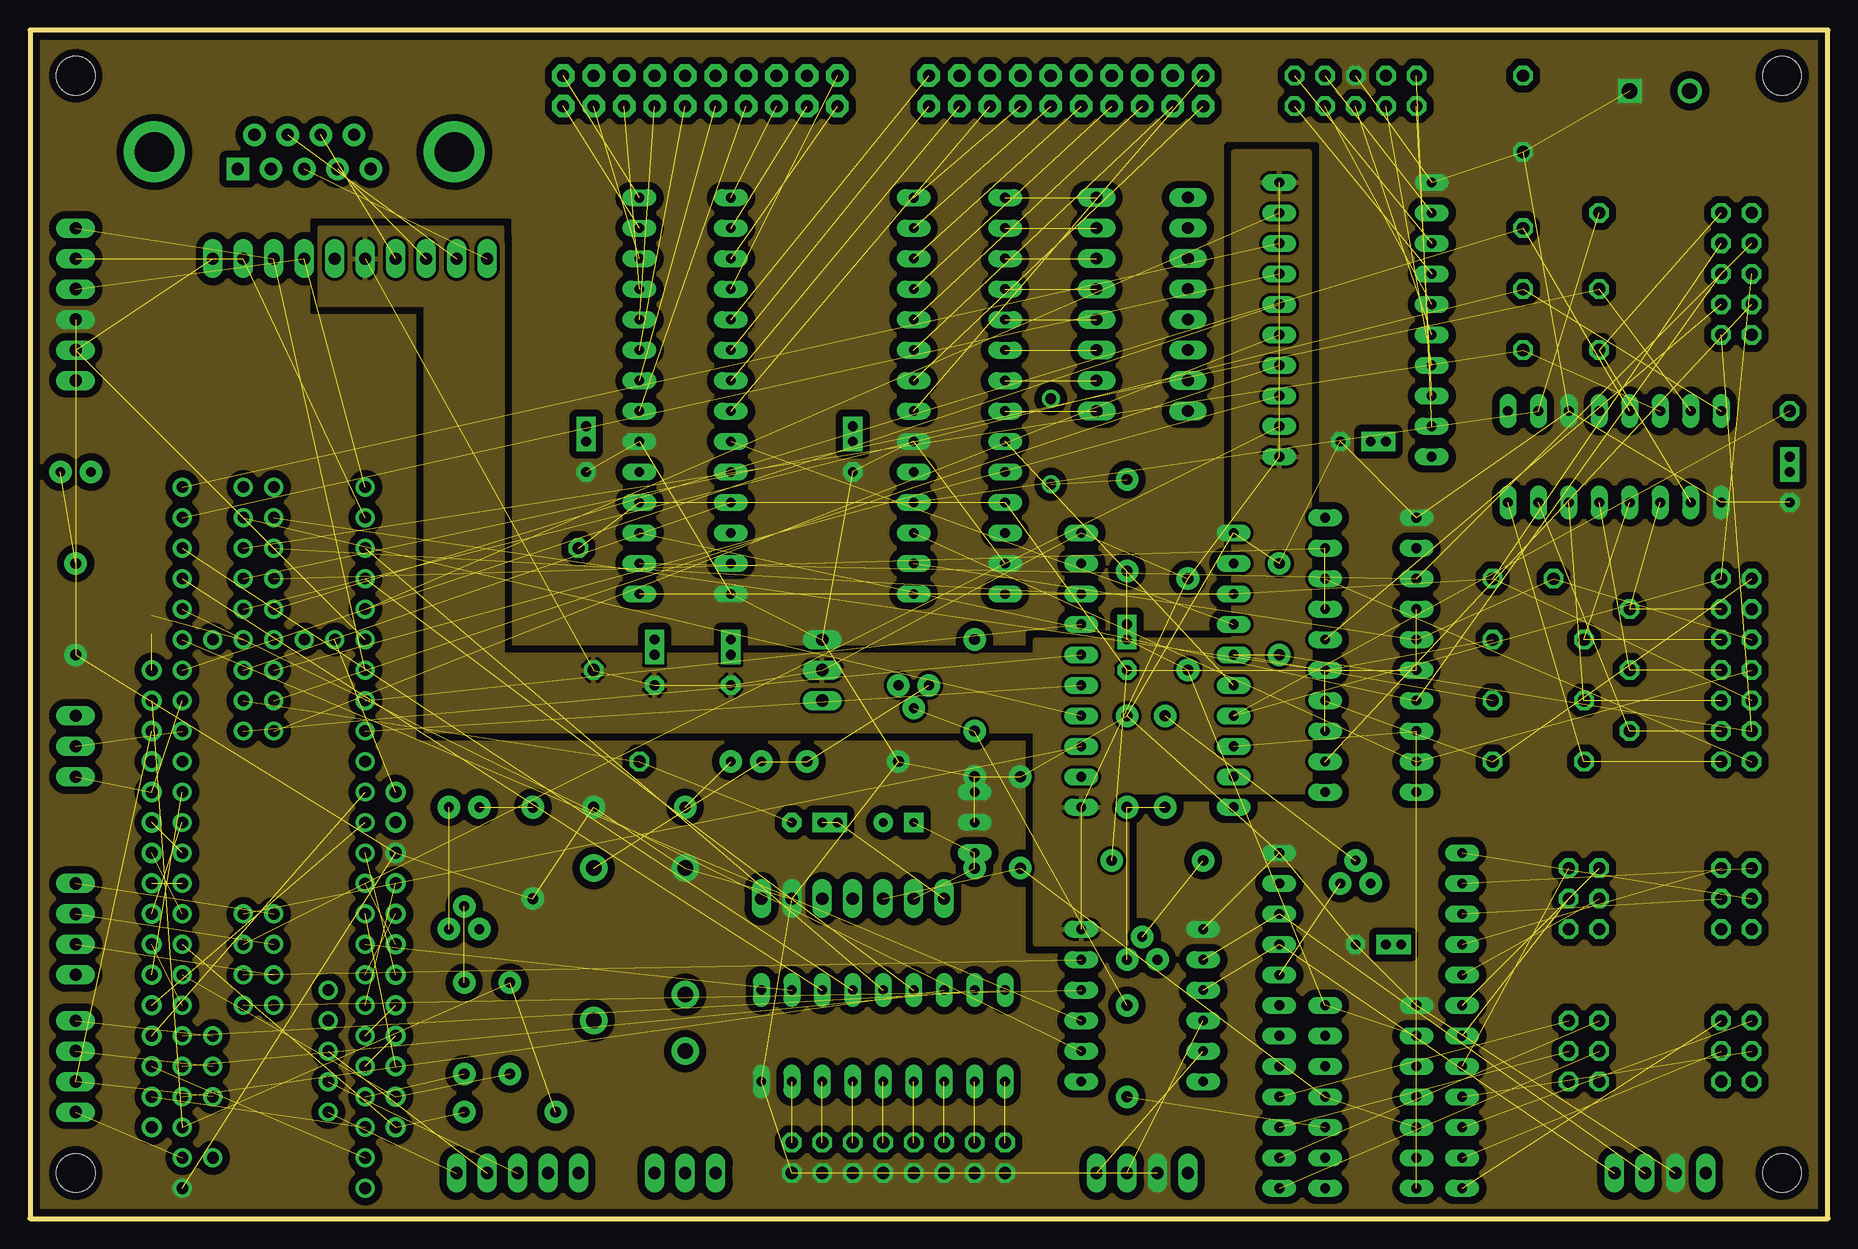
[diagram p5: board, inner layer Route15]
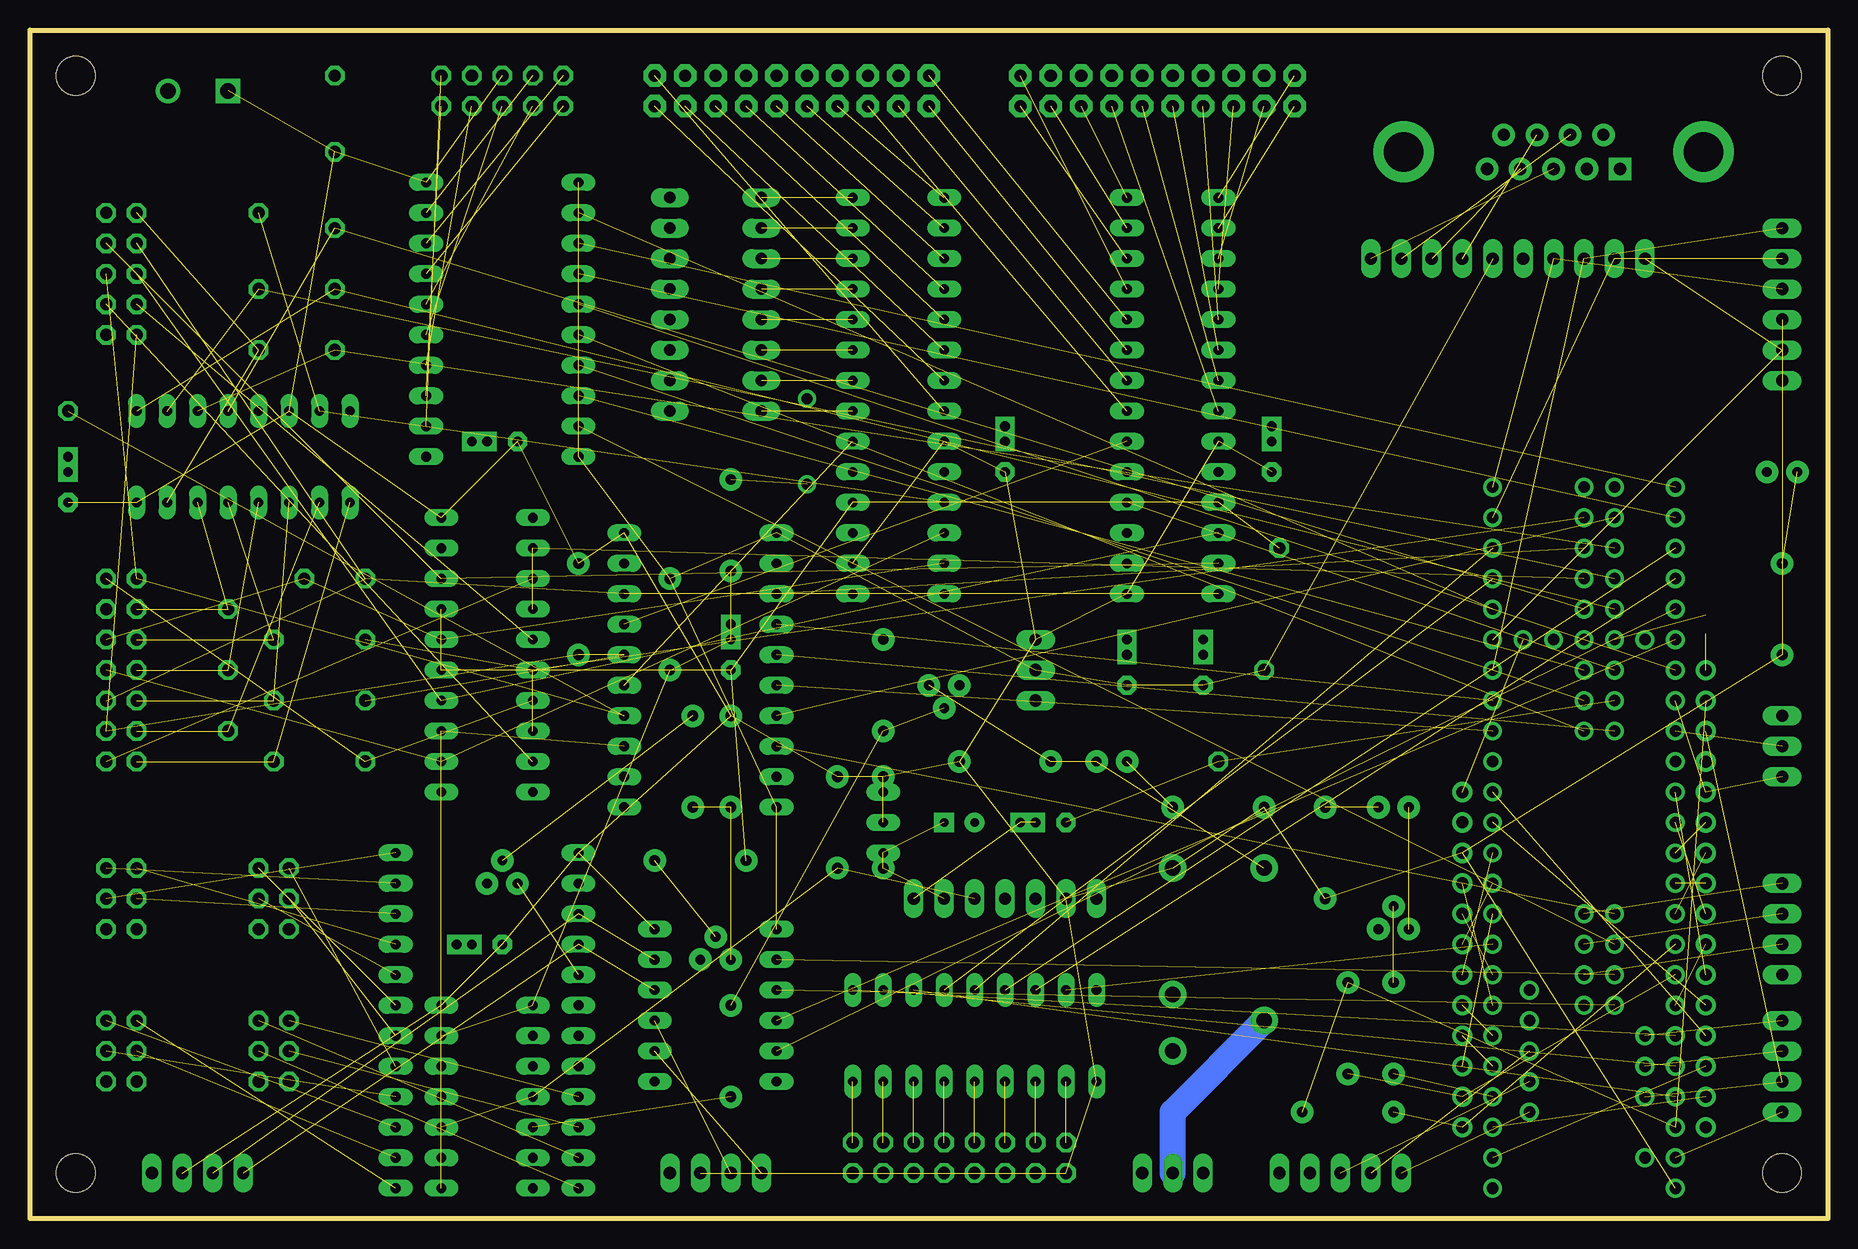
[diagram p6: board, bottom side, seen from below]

Size 149.86 x 99.06 mm. Coordinates in mm from the lower left corner, seen from the top.
Outline: 0,0 149.86,0 149.86,99.06 0,99.06 0,0
Copper layers (1*2*15*16): Top 0.035mm / dielectric 1.5mm / Route2 0.035mm / dielectric 0.15mm / Route15 0.035mm / dielectric 0.2mm / Bottom 0.035mm
Design rules "SparkFun *": minimum track width 8mil, minimum drill 20mil, track to track 8mil, track to pad 8mil, pad to pad 8mil, via to via 8mil, smd to smd 8mil, copper to edge 10mil, drill to drill 8mil, minimum pad ring 12mil, minimum via ring 10mil, stop-mask expansion 4mil, vias tented up to drill 25mil, thermal gap 10mil
Holes 3.2 mm at 3.81,95.25 3.81,3.81 146.05,95.25 146.05,3.81

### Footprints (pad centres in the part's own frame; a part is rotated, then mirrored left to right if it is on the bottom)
B64Y = drill 0.813 long: A 2.54,0; E -2.54,0; S 0,0
1X04 = drill 1.016 long: 1 -3.81,0; 2 -1.27,0; 3 1.27,0; 4 3.81,0
2X10 = drill 1.016 pad 1.88 octagon: 1 -11.43,-1.27; 2 -11.43,1.27; 3 -8.89,-1.27; 4 -8.89,1.27; 5 -6.35,-1.27; 6 -6.35,1.27; 7 -3.81,-1.27; 8 -3.81,1.27; 9 -1.27,-1.27; 10 -1.27,1.27; 11 1.27,-1.27; 12 1.27,1.27; 13 3.81,-1.27; 14 3.81,1.27; 15 6.35,-1.27; 16 6.35,1.27; 17 8.89,-1.27; 18 8.89,1.27; 19 11.43,-1.27; 20 11.43,1.27
DIL20W = drill 0.813 long: 1 -11.43,-6.35; 2 -8.89,-6.35; 3 -6.35,-6.35; 4 -3.81,-6.35; 5 -1.27,-6.35; 6 1.27,-6.35; 7 3.81,-6.35; 8 6.35,-6.35; 9 8.89,-6.35; 10 11.43,-6.35; 11 11.43,6.35; 12 8.89,6.35; 13 6.35,6.35; 14 3.81,6.35; 15 1.27,6.35; 16 -1.27,6.35; 17 -3.81,6.35; 18 -6.35,6.35; 19 -8.89,6.35; 20 -11.43,6.35
DIL12W = drill 0.813 long: 1 -12.7,-5.08; 2 -10.16,-5.08; 3 -7.62,-5.08; 4 -5.08,-5.08; 5 -2.54,-5.08; 6 0,-5.08; 7 0,5.08; 8 -2.54,5.08; 9 -5.08,5.08; 10 -7.62,5.08; 11 -10.16,5.08; 12 -12.7,5.08
DIL24W = drill 0.813 long: 1 -13.97,-7.62; 2 -11.43,-7.62; 3 -8.89,-7.62; 4 -6.35,-7.62; 5 -3.81,-7.62; 6 -1.27,-7.62; 7 1.27,-7.62; 8 3.81,-7.62; 9 6.35,-7.62; 10 8.89,-7.62; 11 11.43,-7.62; 12 13.97,-7.62; 13 13.97,7.62; 14 11.43,7.62; 15 8.89,7.62; 16 6.35,7.62; 17 3.81,7.62; 18 1.27,7.62; 19 -1.27,7.62; 20 -3.81,7.62; 21 -6.35,7.62; 22 -8.89,7.62; 23 -11.43,7.62; 24 -13.97,7.62
1X10 = drill 1.016 long: 1 -11.43,0; 2 -8.89,0; 3 -6.35,0; 4 -3.81,0; 5 -1.27,0; 6 1.27,0; 7 3.81,0; 8 6.35,0; 9 8.89,0; 10 11.43,0
1X01 = drill 1.016 octagon: 1 0,0
1+2CAP = drill 0.813 pad 1.6 octagon: 1 -2.54,0 | drill 0.813 pad 1.6 square: 2@1 0,0; 2@2 1.27,0
CPOL-RADIAL-100UF-25V = drill 0.7 pad 1.651 square: 1 1.27,0 | drill 0.7 pad 1.651: 2 -1.27,0
DIODE-1N4148 = drill 0.9 pad 1.88: A -3.81,0; C 3.81,0
LED5MM = drill 0.813 pad 1.88: A -1.27,0; K 1.27,0
DIODE-ZENER = drill 0.9: P$1 -3.556,0; P$2 3.556,0
1X03 = drill 1.016 long: 1 -2.54,0; 2 0,0; 3 2.54,0
DB9_MALE = drill 1.016 pad 1.88: 1 5.54,-1.42; 2 2.77,-1.42; 3 0,-1.42; 4 -2.77,-1.42; 6 4.15,1.42; 7 1.38,1.42; 8 -1.38,1.42; 9 -4.15,1.42 | drill 1.016 pad 1.88 square: 5 -5.54,-1.42 | drill 3.302 pad 5.08: G1 -12.5,0; G2 12.5,0
1X06 = drill 1.016 long: 1 -6.35,0; 2 -3.81,0; 3 -1.27,0; 4 1.27,0; 5 3.81,0; 6 6.35,0
2X05 = drill 1.016 octagon: 1 -5.08,-1.27; 2 -5.08,1.27; 3 -2.54,-1.27; 4 -2.54,1.27; 5 0,-1.27; 6 0,1.27; 7 2.54,-1.27; 8 2.54,1.27; 9 5.08,-1.27; 10 5.08,1.27
2X03 = drill 1.016 octagon: 1 -2.54,-1.27; 2 -2.54,1.27; 3 0,-1.27; 4 0,1.27; 5 2.54,-1.27; 6 2.54,1.27
DIL16 = drill 0.813 long: 1 -8.89,-3.81; 2 -6.35,-3.81; 3 -3.81,-3.81; 4 -1.27,-3.81; 5 1.27,-3.81; 6 3.81,-3.81; 7 6.35,-3.81; 8 8.89,-3.81; 9 8.89,3.81; 10 6.35,3.81; 11 3.81,3.81; 12 1.27,3.81; 13 -1.27,3.81; 14 -3.81,3.81; 15 -6.35,3.81; 16 -8.89,3.81
DIL14 = drill 0.813 long: 1 -7.62,-3.81; 2 -5.08,-3.81; 3 -2.54,-3.81; 4 0,-3.81; 5 2.54,-3.81; 6 5.08,-3.81; 7 7.62,-3.81; 8 7.62,3.81; 9 5.08,3.81; 10 2.54,3.81; 11 0,3.81; 12 -2.54,3.81; 13 -5.08,3.81; 14 -7.62,3.81
DIL28-3 = drill 0.813 long: 1 -16.51,-3.81; 2 -13.97,-3.81; 3 -11.43,-3.81; 4 -8.89,-3.81; 5 -6.35,-3.81; 6 -3.81,-3.81; 7 -1.27,-3.81; 8 1.27,-3.81; 9 3.81,-3.81; 10 6.35,-3.81; 11 8.89,-3.81; 12 11.43,-3.81; 13 13.97,-3.81; 14 16.51,-3.81; 15 16.51,3.81; 16 13.97,3.81; 17 11.43,3.81; 18 8.89,3.81; 19 6.35,3.81; 20 3.81,3.81; 21 1.27,3.81; 22 -1.27,3.81; 23 -3.81,3.81; 24 -6.35,3.81; 25 -8.89,3.81; 26 -11.43,3.81; 27 -13.97,3.81; 28 -16.51,3.81
DIL20 = drill 0.813 long: 1 -11.43,-3.81; 2 -8.89,-3.81; 3 -6.35,-3.81; 4 -3.81,-3.81; 5 -1.27,-3.81; 6 1.27,-3.81; 7 3.81,-3.81; 8 6.35,-3.81; 9 8.89,-3.81; 10 11.43,-3.81; 11 11.43,3.81; 12 8.89,3.81; 13 6.35,3.81; 14 3.81,3.81; 15 1.27,3.81; 16 -1.27,3.81; 17 -3.81,3.81; 18 -6.35,3.81; 19 -8.89,3.81; 20 -11.43,3.81
SCREWTERMINAL-5MM-2 = drill 1.3 pad 2.032 square: 1 0,0 | drill 1.3 pad 2.032: 2 5,0
2X07 = drill 1.016 octagon: 1 -7.62,-1.27; 2 -7.62,1.27; 3 -5.08,-1.27; 4 -5.08,1.27; 5 -2.54,-1.27; 6 -2.54,1.27; 7 0,-1.27; 8 0,1.27; 9 2.54,-1.27; 10 2.54,1.27; 11 5.08,-1.27; 12 5.08,1.27; 13 7.62,-1.27; 14 7.62,1.27
1X16_ROUND = drill 1 pad 1.676: 1 -19.05,0; 2 -16.51,0; 3 -13.97,0; 4 -11.43,0; 5 -8.89,0; 6 -6.35,0; 7 -3.81,0; 8 -1.27,0; 9 1.27,0; 10 3.81,0; 11 6.35,0; 12 8.89,0; 13 11.43,0; 14 13.97,0; 15 16.51,0; 16 19.05,0
1X12_ROUND = drill 1 pad 1.676: 1 -13.97,0; 2 -11.43,0; 3 -8.89,0; 4 -6.35,0; 5 -3.81,0; 6 -1.27,0; 7 1.27,0; 8 3.81,0; 9 6.35,0; 10 8.89,0; 11 11.43,0; 12 13.97,0
RELAY-JZC = drill 1.3 pad 2.286: 1 3.81,-8.89; 2 -3.81,1.651; 3 -3.81,6.35; 4 3.81,3.81; 5 -3.81,-8.89
2X08 = drill 1.016 octagon: 1 -8.89,-1.27; 2 -8.89,1.27; 3 -6.35,-1.27; 4 -6.35,1.27; 5 -3.81,-1.27; 6 -3.81,1.27; 7 -1.27,-1.27; 8 -1.27,1.27; 9 1.27,-1.27; 10 1.27,1.27; 11 3.81,-1.27; 12 3.81,1.27; 13 6.35,-1.27; 14 6.35,1.27; 15 8.89,-1.27; 16 8.89,1.27
TO-92 = drill 0.813 pad 1.88: 1 -1.27,0; 2 0,1.905; 3 1.27,0
AXIAL-0.3 = drill 0.9 pad 1.88: P$1 -3.81,0; P$2 3.81,0
SOLDERJUMPER_CLOSEDWIRE = smd 1.168 x 1.6: 1 -0.762,0; 2 0.762,0 | smd 0.635 x 0.203: WIRE 0,0
DIPSWITCH-08 = drill 0.97 long: 1 -8.89,-3.81; 2 -6.35,-3.81; 3 -3.81,-3.81; 4 -1.27,-3.81; 5 1.27,-3.81; 6 3.81,-3.81; 7 6.35,-3.81; 8 8.89,-3.81; 9 8.89,3.81; 10 6.35,3.81; 11 3.81,3.81; 12 1.27,3.81; 13 -1.27,3.81; 14 -3.81,3.81; 15 -6.35,3.81; 16 -8.89,3.81
1X07 = drill 1.016 long: 1 -7.62,0; 2 -5.08,0; 3 -2.54,0; 4 0,0; 5 2.54,0; 6 5.08,0; 7 7.62,0
TEENSY-3.6_FULL = drill 0.965: 0 -7.62,5.08; 1 -7.62,2.54; 2 -7.62,0; 3 -7.62,-2.54; 3.3V_2 -2.54,-38.1; 3V3_1 -7.62,-27.94; 3V3_3 2.54,-50.8; 3V3_MAX_250 7.62,2.54; 4 -7.62,-5.08; 5 -7.62,-7.62; 6 -7.62,-10.16; 7 -7.62,-12.7; 8 -7.62,-15.24; 9 -7.62,-17.78; 10 -7.62,-20.32; 11 -7.62,-22.86; 12 -7.62,-25.4; 13 7.62,-25.4; 14 7.62,-22.86; 15 7.62,-20.32; 16 7.62,-17.78; 17 7.62,-15.24; 18 7.62,-12.7; 19 7.62,-10.16; 20 7.62,-7.62; 21 7.62,-5.08; 22 7.62,-2.54; 23 7.62,0; 24 -7.62,-30.48; 25 -7.62,-33.02; 26 -7.62,-35.56; 27 -7.62,-38.1; 28 -7.62,-40.64; 29 -7.62,-43.18; 30 -7.62,-45.72; 31 -7.62,-48.26; 32 -7.62,-50.8; 33 7.62,-50.8; 34 7.62,-48.26; 35 7.62,-45.72; 36 7.62,-43.18; 37 7.62,-40.64; 38 7.62,-38.1; 39 7.62,-35.56; 40 0,-30.48; 41 0,-33.02; 42 0,-35.56; 43 0,-40.64; 44 0,-43.18; 45 0,-45.72; 46 0,-48.26; 47 2.54,-48.26; 48 2.54,-45.72; 49 2.54,-43.18; 50 2.54,-40.64; 51 2.54,-35.56; 52 2.54,-33.02; 53 2.54,-30.48; 54 2.54,-15.24; 55 2.54,-12.7; 56 2.54,-10.16; 57 2.54,-7.62; +5V -4.547,1.27; A10 5.08,-2.54; A11 5.08,-5.08; A21 7.62,-33.02; A22 7.62,-30.48; AGND 7.62,5.08; AREF 5.08,0; D+ -4.547,-3.81; D- -4.547,-1.27; DC 0,-12.7; DD 0,-15.24; DE 0,-10.16; GND1 -7.62,7.62; GND2 7.62,-27.94; GND3 -4.547,-6.35; GND4 -4.547,-8.89; GND5 0,-38.1; GND6 0,-7.62; GND7 0,-50.8; PROGRAM 2.54,-38.1; RESET 5.08,-38.1; VBAT -5.08,-38.1; VIN 7.62,7.62; VUSB 5.08,5.08
DIL18 = drill 0.813 long: 1 -10.16,-3.81; 2 -7.62,-3.81; 3 -5.08,-3.81; 4 -2.54,-3.81; 5 0,-3.81; 6 2.54,-3.81; 7 5.08,-3.81; 8 7.62,-3.81; 9 10.16,-3.81; 10 10.16,3.81; 11 7.62,3.81; 12 5.08,3.81; 13 2.54,3.81; 14 0,3.81; 15 -2.54,3.81; 16 -5.08,3.81; 17 -7.62,3.81; 18 -10.16,3.81
1X05 = drill 1.016 long: 1 -5.08,0; 2 -2.54,0; 3 0,0; 4 2.54,0; 5 5.08,0

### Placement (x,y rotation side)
_  78.74,33.02 90 top
AIN  3.81,12.7 90 top
BANK0  55.88,93.98 0 top
BANK1  86.36,93.98 0 top
BOB1  93.98,45.72 270 top
BOB2  92.71,11.43 270 top
BOB3  111.76,16.51 270 top
BOB4  110.49,74.93 270 top
BOB5  26.67,80.01 180 top
BS0  130.81,72.39 0 top
BS1  133.35,50.8 0 top
BS2  129.54,48.26 0 top
BS3  133.35,45.72 0 top
BS4  129.54,43.18 0 top
BS5  133.35,40.64 0 top
BS6  129.54,38.1 0 top
BS7  45.72,55.88 0 top
C1  68.58,64.77 90 top
C2  113.03,22.86 0 top
C3  66.04,33.02 0 top
C4  52.07,46.99 90 top
C5  58.42,46.99 90 top
C6  72.39,33.02 0 top
C7  46.35,64.77 90 top
C8  91.44,48.26 90 top
C9  146.69,62.23 90 top
C10  111.76,64.77 0 top
CS  124.46,82.55 0 top
CSA0  124.46,77.47 0 top
CSA1  130.81,77.47 0 top
CSA2  124.46,72.39 0 top
D1  68.58,38.1 0 top
D2  59.69,38.1 0 top
D3  3.81,62.23 0 top
D4  85.09,64.77 90 top
DAC  3.81,39.37 270 top
DB9M  22.86,88.9 0 top
DEBUG  3.81,24.13 90 top
FRAME1  0,1.27 0 top
FRAME2  120.65,5.08 0 top
FRAME3  not placed on the board
FTDI  3.81,76.2 90 top
GND  124.46,95.25 0 top
GPIO  110.49,93.98 0 top
I2C1  92.71,3.81 0 top
I2C3  135.89,3.81 0 top
I2C3_0-1  129.54,13.97 270 top
I2C3_2-3  142.24,13.97 270 top
I2C3_4-5  129.54,26.67 270 top
I2C3_6-7  142.24,26.67 270 top
IC1  132.08,63.5 180 top
IC2  111.76,10.16 270 top
IC3  77.47,68.58 270 top
IC4  54.61,68.58 270 top
IC5  111.76,46.99 270 top
IRQ  121.92,43.18 0 top
J2  133.35,93.98 0 top
J238  146.69,67.31 0 top
JP1  142.24,45.72 270 top
JP2  142.24,78.74 270 top
JP3  10.16,26.67 90 top
JP4  30.48,21.59 270 top
K0  50.8,20.32 180 top
LD1117V33  66.04,45.72 90 top
LED  36.2,34.29 180 top
MISO  121.92,53.34 0 top
MOSI  127,53.34 0 top
PWM  72.39,5.08 180 top
Q1  73.66,44.45 180 top
Q2  36.2,24.13 0 top
Q3  92.71,21.59 0 top
Q4  110.49,27.94 0 top
R1  78.74,33.02 90 top
R2  82.55,33.02 90 top
R3  78.74,44.45 270 top
R4  91.44,13.97 270 top
R5  50.8,34.29 180 top
R6  3.81,50.8 270 top
R7  36.2,15.88 270 top
R8  40.01,15.88 90 top
R9  41.91,30.48 270 top
R10  40.01,8.89 0 top
R11  96.52,49.53 90 top
R12  93.98,29.84 180 top
R13  94.61,38.1 270 top
R14  91.44,38.1 270 top
R15  91.44,57.78 90 top
R16  104.14,50.8 270 top
RST  130.81,83.82 0 top
SJ1  10.16,49.53 90 top
SPICLK  121.92,48.26 0 top
SW1  92.71,76.2 90 top
TA8030S  68.58,26.67 180 top
U$1  20.32,10.16 180 top
ULN2308  71.12,15.24 180 top
USB  40.64,3.81 0 top
V3.3  46.99,45.72 0 top
VCC  124.46,88.9 0 top
WD  54.61,3.81 0 top
WD_  121.92,38.1 0 top
WDRFSH  50.8,38.1 0 top

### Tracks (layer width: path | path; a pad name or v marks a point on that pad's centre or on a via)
3  (1 unrouted)
3V3_MAX_250  (3 unrouted)
4  (1 unrouted)
5  (1 unrouted)
6  (1 unrouted)
8  (1 unrouted)
9  (1 unrouted)
10  (1 unrouted)
24  (1 unrouted)
25  (1 unrouted)
28  (1 unrouted)
33  (1 unrouted)
34  (1 unrouted)
39  (1 unrouted)
40  (1 unrouted)
41  (1 unrouted)
42  (1 unrouted)
55  (1 unrouted)
+3V3  (10 unrouted)
  pour Route15: 64.77,46.99 91.44,46.99 91.44,41.91 64.77,41.91
  pour Route15: 100.33,88.9 100.33,39.37 106.68,39.37 106.68,88.9
  pour Route15: 91.44,22.86 83.82,22.86 83.82,48.26 106.68,48.26 106.68,35.56 91.44,35.56
  pour Route15: 33.02,46.99 86.36,46.99 86.36,40.64 33.02,40.64
  pour Route15: 39.37,44.45 39.37,82.55 24.13,82.55 24.13,76.2 33.02,76.2 33.02,44.45
  pour Route15: 39.37,81.28 39.37,44.45 33.02,44.45 33.02,76.2
A0  (1 unrouted)
A1  (1 unrouted)
A2  (1 unrouted)
A3  (1 unrouted)
A6  (1 unrouted)
ADC+  (1 unrouted)
ADC-  (1 unrouted)
AGND  (1 unrouted)
AREF  (2 unrouted)
BS0  (2 unrouted)
BS1  (2 unrouted)
BS2  (2 unrouted)
BS3  (2 unrouted)
BS4  (2 unrouted)
BS5  (2 unrouted)
BS6  (2 unrouted)
BS7  (4 unrouted)
CS2  (2 unrouted)
CSA0  (2 unrouted)
CSA1  (2 unrouted)
CSA2  (2 unrouted)
CTS4  (2 unrouted)
DAC0  (2 unrouted)
DAC1  (1 unrouted)
DI_RESET  (1 unrouted)
DI_WD_LATCH  (2 unrouted)
DIMOSI  (3 unrouted)
DISCK  (2 unrouted)
DO_RESET  (1 unrouted)
DO_WD_LATCH  (1 unrouted)
DOMOSI  (2 unrouted)
DOSCK  (2 unrouted)
GND
  pour Route2 (no thermals): 0,99.06 149.86,99.06 149.86,0 0,0
GP3A0  (1 unrouted)
GP3A1  (1 unrouted)
GP3A2  (1 unrouted)
GP3A3  (1 unrouted)
GP3A4  (1 unrouted)
GP3A5  (1 unrouted)
GP3A6  (1 unrouted)
GP3A7  (1 unrouted)
GP3B0  (1 unrouted)
GP3B1  (1 unrouted)
GP3B2  (1 unrouted)
GP3B3  (1 unrouted)
GP3B4  (1 unrouted)
GP3B5  (1 unrouted)
GP3B6  (1 unrouted)
GP3B7  (1 unrouted)
GP4A0  (1 unrouted)
GP4A1  (1 unrouted)
GP4A2  (1 unrouted)
GP4A3  (1 unrouted)
GP4A4  (1 unrouted)
GP4A5  (1 unrouted)
GP4A6  (1 unrouted)
GP4A7  (1 unrouted)
GP4B0  (1 unrouted)
GP4B1  (1 unrouted)
GP4B2  (1 unrouted)
GP4B3  (1 unrouted)
GP4B4  (1 unrouted)
GP4B5  (1 unrouted)
GP4B6  (1 unrouted)
GP4B7  (1 unrouted)
GPIO28  (1 unrouted)
GPIO33  (1 unrouted)
GPIO34  (1 unrouted)
GPIO39  (1 unrouted)
GPIO40  (1 unrouted)
GPIO41  (1 unrouted)
GPIO42  (1 unrouted)
GPIO55  (1 unrouted)
HRTBT  (1 unrouted)
I2CRESET  (1 unrouted)
INTA3  (1 unrouted)
INTA4  (1 unrouted)
IRQ  (1 unrouted)
IRQ5V  (4 unrouted)
J2_38  (1 unrouted)
J2_38_5  (3 unrouted)
MISO0  (1 unrouted)
MISO2  (1 unrouted)
MISO5  (5 unrouted)
MOSI0  (1 unrouted)
MOSI2  (2 unrouted)
N$2  (1 unrouted)
N$3  (2 unrouted)
N$4  (3 unrouted)
N$5  (2 unrouted)
N$6  (3 unrouted)
N$9  (1 unrouted)
N$11  (2 unrouted)
N$12  (1 unrouted)
N$13  (1 unrouted)
N$14
  Bottom 2.184: WD.2 54.61,8.89 K0.4
N$15
  Top 2.184: K0.3 57.15,11.43 WD.3
N$16  (2 unrouted)
N$17  (2 unrouted)
N$23  (1 unrouted)
N$24  (1 unrouted)
N$25  (1 unrouted)
N$26  (1 unrouted)
N$27  (1 unrouted)
N$28  (1 unrouted)
N$29  (1 unrouted)
N$30  (1 unrouted)
N$32  (1 unrouted)
N$33  (1 unrouted)
N$34  (1 unrouted)
N$35  (1 unrouted)
N$36  (1 unrouted)
N$37  (1 unrouted)
N$38  (1 unrouted)
N$39  (1 unrouted)
N$41  (1 unrouted)
N$42  (1 unrouted)
N$43  (1 unrouted)
N$46  (1 unrouted)
N$47  (1 unrouted)
N$48  (1 unrouted)
NC
  Top 2.184: WD.1 50.8,5.08 50.8,16.51 52.96,18.67 K0.2
PROGRAM  (1 unrouted)
PWM7  (1 unrouted)
PWM21  (1 unrouted)
PWM22  (1 unrouted)
PWM23  (1 unrouted)
PWM29  (1 unrouted)
PWM30  (1 unrouted)
PWM35  (1 unrouted)
PWM36  (1 unrouted)
RESET  (6 unrouted)
RESETWD  (5 unrouted)
RST1  (3 unrouted)
RST/BOOT  (1 unrouted)
RTS4  (2 unrouted)
RX1  (1 unrouted)
RX4  (2 unrouted)
SC0  (1 unrouted)
SC1  (1 unrouted)
SC2  (1 unrouted)
SC3  (1 unrouted)
SC4  (1 unrouted)
SC5  (1 unrouted)
SC6  (1 unrouted)
SC7  (1 unrouted)
SCK0  (1 unrouted)
SCK2  (3 unrouted)
SCL0  (2 unrouted)
SCL1  (1 unrouted)
SCL1_5V  (1 unrouted)
SCL3  (1 unrouted)
SD0  (1 unrouted)
SD1  (1 unrouted)
SD2  (1 unrouted)
SD3  (1 unrouted)
SD4  (1 unrouted)
SD5  (1 unrouted)
SD6  (1 unrouted)
SD7  (1 unrouted)
SDA0  (2 unrouted)
SDA1  (1 unrouted)
SDA1_5V  (1 unrouted)
SDA3  (1 unrouted)
TX1  (1 unrouted)
TX4  (2 unrouted)
VBAT  (1 unrouted)
VCC  (46 unrouted)
  pour Route15 (isolate 0.61, rank 3, no thermals): 0,99.06 149.86,99.06 149.86,0 0,0
WD_LATCH_3  (1 unrouted)
WD_LATCH_5  (3 unrouted)
WD_RFSH  (2 unrouted)
WDOUT  (1 unrouted)

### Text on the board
tPlace: 20 | 20 | 10 | 1 | 1 | 1 | +5V | gnd | TX4/Rx4 | RTS | BS0 | RxD | MISO | MOSI | TxD | SCK | J238 | Vcc | RST | WD | CTS | IRQ | Gnd | R2Out | R1Out | T2In | T1In | Gnd | Vcc | R2In | R1In | T2Out | T1Out | Gnd | CTS | RxD | RTS | TxD | Pwr | J238 | WD | vcc | BS1 | Gnd | BS2 | MOSI | 3.3v | BS3 | SCK | BS4 | MISO | 1 | G | Weensy 3.6 / Copyright 2017 / Plantation / Productions, Inc. / Rev 4 | BS5 | IRQ | 1 | BS6 | RST | 0 | SD4 | SD5 | SD6 | SD7 | SC4 | SC5 | SC6 | SC7 | 1 | Gnd | Gnd | Gnd | Gnd | A0- | SD0 | SD1 | SD2 | SD3 | A0+ | SC0 | SC1 | SC2 | SC3 | AR | Gnd | Gnd | Gnd | Gnd | AG | 1 | NC | COM | NO | SCL | SDA | +5V | Gnd | SCL | SDA | +5V | Gnd | 16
